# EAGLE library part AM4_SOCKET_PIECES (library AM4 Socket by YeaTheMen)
AM4 Socket Pins broken down into individual sections for convienience. Though it wasnt convientient for me as i spent hours making it >:I by yours truly, YeaTheMen
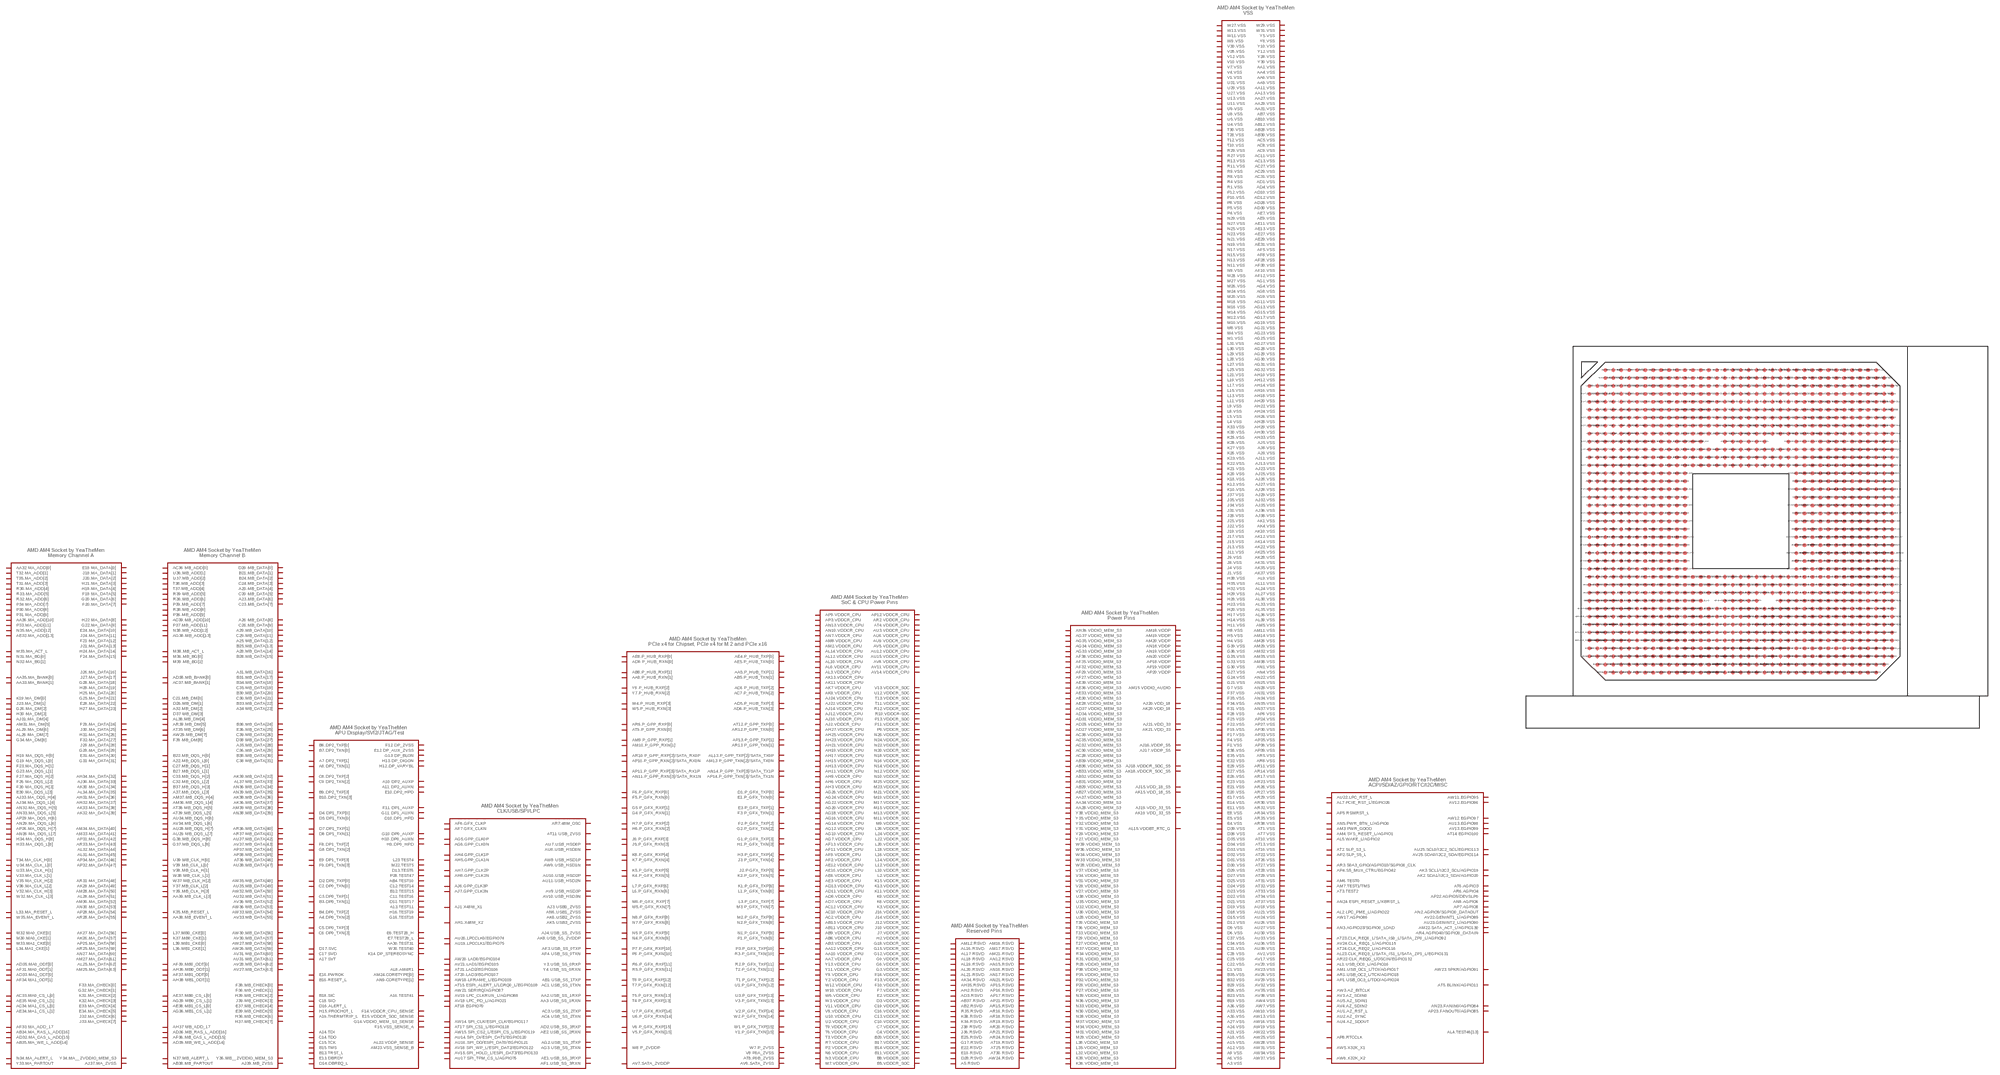
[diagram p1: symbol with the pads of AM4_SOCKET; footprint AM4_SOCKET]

Designator prefix -; gates G$1=AM4_SOCKET_MEM_A G$2=AM4_SOCKET_MEM_B G$3=AM4_SOCKET_CONTROL G$4=AM4_SOCKET_IO G$5=AM4_SOCKET_PCIE G$6=AM4_SOCKET_PWR G$7=AM4_SOCKET_RSVD G$8=AM4_SOCKET_VDD G$9=AM4_SOCKET_VSS G$10=AM4_SOCKET_MISC

## AM4_SOCKET_PIECES  [AM4_SOCKET]
A3.VSS  G$9:A3.VSS  out
A4.DP0_TXN[2]  G$3:A4.DP0_TXN[2]
A5.RSVD  G$7:A5.RSVD  nc
A6.VSS  G$9:A6.VSS  out
A7.DP2_TXP[1]  G$3:A7.DP2_TXP[1]
A8.DP2_TXN[1]  G$3:A8.DP2_TXN[1]
A9.VSS  G$9:A9.VSS  out
A10.DP2_AUXP  G$3:A10.DP2_AUXP
A11.DP2_AUXN  G$3:A11.DP2_AUXN
A12.VSS  G$9:A12.VSS  out
A13.TEST11  G$3:A13.TEST11
A14.TDI  G$3:A14.TDI
A15.VSS  G$9:A15.VSS  out
A16.TEST41  G$3:A16.TEST41
A17.SVT  G$3:A17.SVT
A18.VSS  G$9:A18.VSS  out
A19.THERMTRIP_L  G$3:A19.THERMTRIP_L
A20.MB_DATA[4]  G$2:A20.MB_DATA[4]
A21.VSS  G$9:A21.VSS  out
A22.MB_DQS_L[0]  G$2:A22.MB_DQS_L[0]
A23.MB_DATA[6]  G$2:A23.MB_DATA[6]
A24.VSS  G$9:A24.VSS  out
A25.MB_DATA[12]  G$2:A25.MB_DATA[12]
A26.MB_DATA[8]  G$2:A26.MB_DATA[8]
A27.VSS  G$9:A27.VSS  out
A28.MB_DATA[14]  G$2:A28.MB_DATA[14]
A29.MB_DATA[10]  G$2:A29.MB_DATA[10]
A30.VSS  G$9:A30.VSS  out
A31.MB_DATA[16]  G$2:A31.MB_DATA[16]
A32.MB_DM[2]  G$2:A32.MB_DM[2]
A33.VSS  G$9:A33.VSS  out
A34.MB_DATA[23]  G$2:A34.MB_DATA[23]
A35.MB_DATA[28]  G$2:A35.MB_DATA[28]
A36.VSS  G$9:A36.VSS  out
A37.MB_DQS_L[3]  G$2:A37.MB_DQS_L[3]
AA1.VSS  G$9:AA1.VSS  out
AA2.USB_SS_1RXP  G$4:AA2.USB_SS_1RXP
AA3.USB_SS_1RXN  G$4:AA3.USB_SS_1RXN
AA4.VSS  G$9:AA4.VSS  out
AA5.P_HUB_TXP[1]  G$5:AA5.P_HUB_TXP[1]
AA6.VSS  G$9:AA6.VSS  out
AA7.VDDCR_CPU  G$6:AA7.VDDCR_CPU  pwr
AA8.P_HUB_RXN[1]  G$5:AA8.P_HUB_RXN[1]
AA9.VSS  G$9:AA9.VSS  out
AA10.VDDCR_CPU  G$6:AA10.VDDCR_CPU  pwr
AA11.VSS  G$9:AA11.VSS  out
AA12.VDDCR_CPU  G$6:AA12.VDDCR_CPU  pwr
AA13.VSS  G$9:AA13.VSS  out
AA27.VSS  G$9:AA27.VSS  out
AA28.VDDIO_MEM_S3  G$8:AA28.VDDIO_MEM_S3  pwr
AA29.VSS  G$9:AA29.VSS  out
AA30.TEST31  G$3:AA30.TEST31
AA31.VSS  G$9:AA31.VSS  out
AA32.MA_ADD[0]  G$1:AA32.MA_ADD[0]
AA33.MA_BANK[1]  G$1:AA33.MA_BANK[1]
AA34.VDDIO_MEM_S3  G$8:AA34.VDDIO_MEM_S3  pwr
AA35.MA_BANK[0]  G$1:AA35.MA_BANK[0]
AA36.MA_ADD[10]  G$1:AA36.MA_ADD[10]
AA37.VDDIO_MEM_S3  G$8:AA37.VDDIO_MEM_S3  pwr
AA38.MB_EVENT_L  G$2:AA38.MB_EVENT_L
AA39.MB_CLK_L[3]  G$2:AA39.MB_CLK_L[3]
AB1.USB_SS_1TXP  G$4:AB1.USB_SS_1TXP
AB2.RSVD  G$7:AB2.RSVD  nc
AB3.VDDCR_CPU  G$6:AB3.VDDCR_CPU  pwr
AB4.TEST10  G$3:AB4.TEST10
AB5.P_HUB_TXN[1]  G$5:AB5.P_HUB_TXN[1]
AB6.VDDCR_CPU  G$6:AB6.VDDCR_CPU  pwr
AB7.VSS  G$9:AB7.VSS  out
AB8.P_HUB_RXP[1]  G$5:AB8.P_HUB_RXP[1]
AB9.VDDCR_CPU  G$6:AB9.VDDCR_CPU  pwr
AB10.VSS  G$9:AB10.VSS  out
AB11.VDDCR_CPU  G$6:AB11.VDDCR_CPU  pwr
AB12.VSS  G$9:AB12.VSS  out
AB13.VDDCR_CPU  G$6:AB13.VDDCR_CPU  pwr
AB27.VDDIO_MEM_S3  G$8:AB27.VDDIO_MEM_S3  pwr
AB28.VSS  G$9:AB28.VSS  out
AB29.VDDIO_MEM_S3  G$8:AB29.VDDIO_MEM_S3  pwr
AB30.VSS  G$9:AB30.VSS  out
AB31.VDDIO_MEM_S3  G$8:AB31.VDDIO_MEM_S3  pwr
AB32.VDDIO_MEM_S3  G$8:AB32.VDDIO_MEM_S3  pwr
AB33.VDDIO_MEM_S3  G$8:AB33.VDDIO_MEM_S3  pwr
AB34.MA_RAS_L_ADD[16]  G$1:AB34.MA_RAS_L_ADD[16]
AB35.MA_WE_L_ADD[14]  G$1:AB35.MA_WE_L_ADD[14]
AB36.VDDIO_MEM_S3  G$8:AB36.VDDIO_MEM_S3  pwr
AB37.RSVD  G$7:AB37.RSVD  nc
AB38.MB_PARTOUT  G$2:AB38.MB_PARTOUT  out
AB39.VDDIO_MEM_S3  G$8:AB39.VDDIO_MEM_S3  pwr
AC1.USB_SS_1TXN  G$4:AC1.USB_SS_1TXN
AC2.VDDCR_CPU  G$6:AC2.VDDCR_CPU  pwr
AC3.USB_SS_2TXP  G$4:AC3.USB_SS_2TXP
AC4.USB_SS_2TXN  G$4:AC4.USB_SS_2TXN
AC5.VSS  G$9:AC5.VSS  out
AC6.P_HUB_TXP[2]  G$5:AC6.P_HUB_TXP[2]
AC7.P_HUB_TXN[2]  G$5:AC7.P_HUB_TXN[2]
AC8.VSS  G$9:AC8.VSS  out
AC9.VSS  G$9:AC9.VSS  out
AC10.VDDCR_CPU  G$6:AC10.VDDCR_CPU  pwr
AC11.VSS  G$9:AC11.VSS  out
AC12.VDDCR_CPU  G$6:AC12.VDDCR_CPU  pwr
AC13.VSS  G$9:AC13.VSS  out
AC27.VSS  G$9:AC27.VSS  out
AC28.VDDIO_MEM_S3  G$8:AC28.VDDIO_MEM_S3  pwr
AC29.VSS  G$9:AC29.VSS  out
AC30.VDDIO_MEM_S3  G$8:AC30.VDDIO_MEM_S3  pwr
AC31.VSS  G$9:AC31.VSS  out
AC32.VDDIO_MEM_S3  G$8:AC32.VDDIO_MEM_S3  pwr
AC33.MA0_CS_L[0]  G$1:AC33.MA0_CS_L[0]
AC34.MA1_CS_L[0]  G$1:AC34.MA1_CS_L[0]
AC35.VDDIO_MEM_S3  G$8:AC35.VDDIO_MEM_S3  pwr
AC36.MB_ADD[0]  G$2:AC36.MB_ADD[0]
AC37.MB_BANK[1]  G$2:AC37.MB_BANK[1]
AC38.VDDIO_MEM_S3  G$8:AC38.VDDIO_MEM_S3  pwr
AC39.MB_ADD[10]  G$2:AC39.MB_ADD[10]
AD1.VSS  G$9:AD1.VSS  out
AD2.USB_SS_3RXP  G$4:AD2.USB_SS_3RXP
AD3.RSVD  G$7:AD3.RSVD  nc
AD4.VSS  G$9:AD4.VSS  out
AD5.P_HUB_TXP[3]  G$5:AD5.P_HUB_TXP[3]
AD6.P_HUB_TXN[3]  G$5:AD6.P_HUB_TXN[3]
AD7.VDDCR_CPU  G$6:AD7.VDDCR_CPU  pwr
AD8.P_HUB_RXN[0]  G$5:AD8.P_HUB_RXN[0]
AD9.VDDCR_CPU  G$6:AD9.VDDCR_CPU  pwr
AD10.VSS  G$9:AD10.VSS  out
AD11.VDDCR_CPU  G$6:AD11.VDDCR_CPU  pwr
AD12.VSS  G$9:AD12.VSS  out
AD13.VDDCR_CPU  G$6:AD13.VDDCR_CPU  pwr
AD27.VDDIO_MEM_S3  G$8:AD27.VDDIO_MEM_S3  pwr
AD28.VSS  G$9:AD28.VSS  out
AD29.VDDIO_MEM_S3  G$8:AD29.VDDIO_MEM_S3  pwr
AD30.VSS  G$9:AD30.VSS  out
AD31.VDDIO_MEM_S3  G$8:AD31.VDDIO_MEM_S3  pwr
AD32.MA_CAS_L_ADD[15]  G$1:AD32.MA_CAS_L_ADD[15]
AD33.MA1_ODT[0]  G$1:AD33.MA1_ODT[0]
AD34.VDDIO_MEM_S3  G$8:AD34.VDDIO_MEM_S3  pwr
AD35.MA0_ODT[0]  G$1:AD35.MA0_ODT[0]
AD36.MB_RAS_L_ADD[16]  G$2:AD36.MB_RAS_L_ADD[16]
AD37.VDDIO_MEM_S3  G$8:AD37.VDDIO_MEM_S3  pwr
AD38.MB_BANK[0]  G$2:AD38.MB_BANK[0]
AD39.MB_WE_L_ADD[14]  G$2:AD39.MB_WE_L_ADD[14]
AE1.USB_SS_3RXP  G$4:AE1.USB_SS_3RXP
AE2.USB_SS_2RXN  G$4:AE2.USB_SS_2RXN
AE3.VDDCR_CPU  G$6:AE3.VDDCR_CPU  pwr
AE4.P_HUB_TXP[0]  G$5:AE4.P_HUB_TXP[0]
AE5.P_HUB_TXN[0]  G$5:AE5.P_HUB_TXN[0]
AE6.VDDCR_CPU  G$6:AE6.VDDCR_CPU  pwr
AE7.VSS  G$9:AE7.VSS  out
AE8.P_HUB_RXP[0]  G$5:AE8.P_HUB_RXP[0]
AE9.VSS  G$9:AE9.VSS  out
AE10.VDDCR_CPU  G$6:AE10.VDDCR_CPU  pwr
AE11.VSS  G$9:AE11.VSS  out
AE12.VDDCR_CPU  G$6:AE12.VDDCR_CPU  pwr
AE13.VSS  G$9:AE13.VSS  out
AE27.VSS  G$9:AE27.VSS  out
AE28.VDDIO_MEM_S3  G$8:AE28.VDDIO_MEM_S3  pwr
AE29.VSS  G$9:AE29.VSS  out
AE30.VDDIO_MEM_S3  G$8:AE30.VDDIO_MEM_S3  pwr
AE31.VSS  G$9:AE31.VSS  out
AE32.MA_ADD[13]  G$1:AE32.MA_ADD[13]
AE33.VDDIO_MEM_S3  G$8:AE33.VDDIO_MEM_S3  pwr
AE34.MA1_CS_L[1]  G$1:AE34.MA1_CS_L[1]
AE35.MA0_CS_L[1]  G$1:AE35.MA0_CS_L[1]
AE36.VDDIO_MEM_S3  G$8:AE36.VDDIO_MEM_S3  pwr
AE37.MB0_CS_L[0]  G$2:AE37.MB0_CS_L[0]
AE38.MB1_CS_L[0]  G$2:AE38.MB1_CS_L[0]
AE39.VDDIO_MEM_S3  G$8:AE39.VDDIO_MEM_S3  pwr
AF1.USB_SS_3RXN  G$4:AF1.USB_SS_3RXN
AF2.VDDCR_CPU  G$6:AF2.VDDCR_CPU  pwr
AF3.USB_SS_0TXP  G$4:AF3.USB_SS_0TXP
AF4.USB_SS_0TXN  G$4:AF4.USB_SS_0TXN
AF5.VSS  G$9:AF5.VSS  out
AF6.GFX_CLKP  G$4:AF6.GFX_CLKP
AF7.GFX_CLKN  G$4:AF7.GFX_CLKN
AF8.VSS  G$9:AF8.VSS  out
AF9.VDDCR_CPU  G$6:AF9.VDDCR_CPU  pwr
AF10.VSS  G$9:AF10.VSS  out
AF11.VDDCR_CPU  G$6:AF11.VDDCR_CPU  pwr
AF12.VSS  G$9:AF12.VSS  out
AF13.VDDCR_CPU  G$6:AF13.VDDCR_CPU  pwr
AF27.VDDIO_MEM_S3  G$8:AF27.VDDIO_MEM_S3  pwr
AF28.VSS  G$9:AF28.VSS  out
AF29.VDDIO_MEM_S3  G$8:AF29.VDDIO_MEM_S3  pwr
AF30.VSS  G$9:AF30.VSS  out
AF31.MA0_ODT[1]  G$1:AF31.MA0_ODT[1]
AF32.VDDIO_MEM_S3  G$8:AF32.VDDIO_MEM_S3  pwr
AF33.MA_ADD_17  G$1:AF33.MA_ADD_17
AF34.MA1_ODT[1]  G$1:AF34.MA1_ODT[1]
AF35.VDDIO_MEM_S3  G$8:AF35.VDDIO_MEM_S3  pwr
AF36.MB_CAS_L_ADD[15]  G$2:AF36.MB_CAS_L_ADD[15]
AF37.MB1_ODT[0]  G$2:AF37.MB1_ODT[0]
AF38.VDDIO_MEM_S3  G$8:AF38.VDDIO_MEM_S3  pwr
AF39.MB0_ODT[0]  G$2:AF39.MB0_ODT[0]
AG1.VSS  G$9:AG1.VSS  out
AG2.USB_SS_3TXP  G$4:AG2.USB_SS_3TXP
AG3.USB_SS_3TXN  G$4:AG3.USB_SS_3TXN
AG4.VSS  G$9:AG4.VSS  out
AG5.GPP_CLK0P  G$4:AG5.GPP_CLK0P
AG6.GPP_CLK0N  G$4:AG6.GPP_CLK0N
AG7.VDDCR_CPU  G$6:AG7.VDDCR_CPU  pwr
AG8.VSS  G$9:AG8.VSS  out
AG9.VSS  G$9:AG9.VSS  out
AG10.VDDCR_CPU  G$6:AG10.VDDCR_CPU  pwr
AG11.VSS  G$9:AG11.VSS  out
AG12.VDDCR_CPU  G$6:AG12.VDDCR_CPU  pwr
AG13.VSS  G$9:AG13.VSS  out
AG14.VDDCR_CPU  G$6:AG14.VDDCR_CPU  pwr
AG15.VSS  G$9:AG15.VSS  out
AG16.VDDCR_CPU  G$6:AG16.VDDCR_CPU  pwr
AG17.VSS  G$9:AG17.VSS  out
AG18.VDDCR_CPU  G$6:AG18.VDDCR_CPU  pwr
AG19.VSS  G$9:AG19.VSS  out
AG20.VDDCR_CPU  G$6:AG20.VDDCR_CPU  pwr
AG21.VSS  G$9:AG21.VSS  out
AG22.VDDCR_CPU  G$6:AG22.VDDCR_CPU  pwr
AG23.VSS  G$9:AG23.VSS  out
AG24.VDDCR_CPU  G$6:AG24.VDDCR_CPU  pwr
AG25.VSS  G$9:AG25.VSS  out
AG26.VDDCR_CPU  G$6:AG26.VDDCR_CPU  pwr
AG27.VSS  G$9:AG27.VSS  out
AG28.VSS  G$9:AG28.VSS  out
AG29.VSS  G$9:AG29.VSS  out
AG30.VSS  G$9:AG30.VSS  out
AG31.VSS  G$9:AG31.VSS  out
AG32.VSS  G$9:AG32.VSS  out
AG33.VDDIO_MEM_S3  G$8:AG33.VDDIO_MEM_S3  pwr
AG34.VDDIO_MEM_S3  G$8:AG34.VDDIO_MEM_S3  pwr
AG35.VDDIO_MEM_S3  G$8:AG35.VDDIO_MEM_S3  pwr
AG36.MB1_CS_L[1]  G$2:AG36.MB1_CS_L[1]
AG37.VDDIO_MEM_S3  G$8:AG37.VDDIO_MEM_S3  pwr
AG38.MB_ADD[13]  G$2:AG38.MB_ADD[13]
AG39.MB0_CS_L[1]  G$2:AG39.MB0_CS_L[1]
AH1.X48M_X2  G$4:AH1.X48M_X2
AH2.RSVD  G$7:AH2.RSVD  nc
AH3.VDDCR_CPU  G$6:AH3.VDDCR_CPU  pwr
AH4.GPP_CLK1P  G$4:AH4.GPP_CLK1P
AH5.GPP_CLK1N  G$4:AH5.GPP_CLK1N
AH6.VDDCR_CPU  G$6:AH6.VDDCR_CPU  pwr
AH7.GPP_CLK2P  G$4:AH7.GPP_CLK2P
AH8.GPP_CLK2N  G$4:AH8.GPP_CLK2N
AH9.VDDCR_CPU  G$6:AH9.VDDCR_CPU  pwr
AH10.VSS  G$9:AH10.VSS  out
AH11.VDDCR_CPU  G$6:AH11.VDDCR_CPU  pwr
AH12.VSS  G$9:AH12.VSS  out
AH13.VDDCR_CPU  G$6:AH13.VDDCR_CPU  pwr
AH14.VSS  G$9:AH14.VSS  out
AH15.VDDCR_CPU  G$6:AH15.VDDCR_CPU  pwr
AH16.VSS  G$9:AH16.VSS  out
AH17.VDDCR_CPU  G$6:AH17.VDDCR_CPU  pwr
AH18.VSS  G$9:AH18.VSS  out
AH19.VDDCR_CPU  G$6:AH19.VDDCR_CPU  pwr
AH20.VSS  G$9:AH20.VSS  out
AH21.VDDCR_CPU  G$6:AH21.VDDCR_CPU  pwr
AH22.VSS  G$9:AH22.VSS  out
AH23.VDDCR_CPU  G$6:AH23.VDDCR_CPU  pwr
AH24.VSS  G$9:AH24.VSS  out
AH25.VDDCR_CPU  G$6:AH25.VDDCR_CPU  pwr
AH26.VSS  G$9:AH26.VSS  out
AH27.VDDCR_CPU  G$6:AH27.VDDCR_CPU  pwr
AH28.VSS  G$9:AH28.VSS  out
AH29.VSS  G$9:AH29.VSS  out
AH30.VSS  G$9:AH30.VSS  out
AH31.MA_DATA[36]  G$1:AH31.MA_DATA[36]
AH32.MA_DATA[37]  G$1:AH32.MA_DATA[37]
AH33.VSS  G$9:AH33.VSS  out
AH34.MA_DATA[32]  G$1:AH34.MA_DATA[32]
AH35.RSVD  G$7:AH35.RSVD  nc
AH36.MB0_ODT[1]  G$2:AH36.MB0_ODT[1]
AH37.MB_ADD_17  G$2:AH37.MB_ADD_17
AH38.MB1_ODT[1]  G$2:AH38.MB1_ODT[1]
AH39.VDDIO_MEM_S3  G$8:AH39.VDDIO_MEM_S3  pwr
AJ1.X48M_X1  G$4:AJ1.X48M_X1
AJ2.VDDCR_CPU  G$6:AJ2.VDDCR_CPU  pwr
AJ3.USB0_ZVSS  G$4:AJ3.USB0_ZVSS  out
AJ4.USB_SS_ZVSS  G$4:AJ4.USB_SS_ZVSS  out
AJ5.VSS  G$9:AJ5.VSS  out
AJ6.GPP_CLK3P  G$4:AJ6.GPP_CLK3P
AJ7.GPP_CLK3N  G$4:AJ7.GPP_CLK3N
AJ8.VSS  G$9:AJ8.VSS  out
AJ9.VSS  G$9:AJ9.VSS  out
AJ10.VDDCR_CPU  G$6:AJ10.VDDCR_CPU  pwr
AJ11.VSS  G$9:AJ11.VSS  out
AJ12.VDDCR_CPU  G$6:AJ12.VDDCR_CPU  pwr
AJ13.VSS  G$9:AJ13.VSS  out
AJ14.VDDCR_CPU  G$6:AJ14.VDDCR_CPU  pwr
AJ15.VDD_18_S5  G$8:AJ15.VDD_18_S5  pwr
AJ16.VDDP_S5  G$8:AJ16.VDDP_S5  pwr
AJ17.VDDP_S5  G$8:AJ17.VDDP_S5  pwr
AJ18.VDDCR_SOC_S5  G$8:AJ18.VDDCR_SOC_S5  pwr
AJ19.VDD_33_S5  G$8:AJ19.VDD_33_S5  pwr
AJ20.VDD_18  G$8:AJ20.VDD_18  pwr
AJ21.VDD_33  G$8:AJ21.VDD_33  pwr
AJ22.VDDCR_CPU  G$6:AJ22.VDDCR_CPU  pwr
AJ23.VSS  G$9:AJ23.VSS  out
AJ24.VDDCR_CPU  G$6:AJ24.VDDCR_CPU  pwr
AJ25.VSS  G$9:AJ25.VSS  out
AJ26.VSS  G$9:AJ26.VSS  out
AJ27.VSS  G$9:AJ27.VSS  out
AJ28.VSS  G$9:AJ28.VSS  out
AJ29.VSS  G$9:AJ29.VSS  out
AJ30.MA_DATA[33]  G$1:AJ30.MA_DATA[33]
AJ31.MA_DM[4]  G$1:AJ31.MA_DM[4]
AJ32.VSS  G$9:AJ32.VSS  out
AJ33.MA_DQS_H[4]  G$1:AJ33.MA_DQS_H[4]
AJ34.MA_DQS_L[4]  G$1:AJ34.MA_DQS_L[4]
AJ35.VSS  G$9:AJ35.VSS  out
AJ36.VSS  G$9:AJ36.VSS  out
AJ37.MA_ZVSS  G$1:AJ37.MA_ZVSS  out
AJ38.VSS  G$9:AJ38.VSS  out
AJ39.MB_ZVSS  G$2:AJ39.MB_ZVSS  out
AK1.VSS  G$9:AK1.VSS  out
AK2.SDA1/I2C3_SDA/AGPIO20  G$10:AK2.SDA1/I2C3_SDA/AGPIO20
AK3.SCL1/I2C3_SCL/AGPIO19  G$10:AK3.SCL1/I2C3_SCL/AGPIO19
AK4.VSS  G$9:AK4.VSS  out
AK5.USB3_ZVSS  G$4:AK5.USB3_ZVSS  out
AK6.USB2_ZVSS  G$4:AK6.USB2_ZVSS  out
AK7.VDDCR_CPU  G$6:AK7.VDDCR_CPU  pwr
AK8.USB_SS_ZVDDP  G$4:AK8.USB_SS_ZVDDP  pwr
AK9.VDDCR_CPU  G$6:AK9.VDDCR_CPU  pwr
AK10.VSS  G$9:AK10.VSS  out
AK11.VDDCR_CPU  G$6:AK11.VDDCR_CPU  pwr
AK12.VSS  G$9:AK12.VSS  out
AK13.VDDCR_CPU  G$6:AK13.VDDCR_CPU  pwr
AK14.VSS  G$9:AK14.VSS  out
AK15.VDD_18_S5  G$8:AK15.VDD_18_S5  pwr
AK18.VDDCR_SOC_S5  G$8:AK18.VDDCR_SOC_S5  pwr
AK19.VDD_33_S5  G$8:AK19.VDD_33_S5  pwr
AK20.VDD_18  G$8:AK20.VDD_18  pwr
AK21.VDD_33  G$8:AK21.VDD_33  pwr
AK22.VSS  G$9:AK22.VSS  out
AK25.VSS  G$9:AK25.VSS  out
AK26.MA_DATA[57]  G$1:AK26.MA_DATA[57]
AK27.MA_DATA[56]  G$1:AK27.MA_DATA[56]
AK28.VSS  G$9:AK28.VSS  out
AK29.MA_DATA[49]  G$1:AK29.MA_DATA[49]
AK30.MA_DATA[34]  G$1:AK30.MA_DATA[34]
AK31.VSS  G$9:AK31.VSS  out
AK32.MA_DATA[39]  G$1:AK32.MA_DATA[39]
AK33.MA_DATA[38]  G$1:AK33.MA_DATA[38]
AK34.RSVD  G$7:AK34.RSVD  nc
AK35.VSS  G$9:AK35.VSS  out
AK36.MB_DATA[37]  G$2:AK36.MB_DATA[37]
AK37.VSS  G$9:AK37.VSS  out
AK38.MB_DATA[36]  G$2:AK38.MB_DATA[36]
AK39.MB_DATA[32]  G$2:AK39.MB_DATA[32]
AL1.USB_OC0_L/AGPIO16  G$10:AL1.USB_OC0_L/AGPIO16
AL2.LPC_PME_L/AGPIO22  G$10:AL2.LPC_PME_L/AGPIO22
AL3.VDDCR_CPU  G$6:AL3.VDDCR_CPU  pwr
AL4.TEST46[13]  G$10:AL4.TEST46[13]
AL5.WAKE_L/AGPIO2  G$10:AL5.WAKE_L/AGPIO2
AL6.VDDCR_CPU  G$6:AL6.VDDCR_CPU  pwr
AL7.PCIE_RST_L/EGPIO26  G$10:AL7.PCIE_RST_L/EGPIO26
AL8.AM4R1  G$3:AL8.AM4R1
AL9.VSS  G$9:AL9.VSS  out
AL10.VDDCR_CPU  G$6:AL10.VDDCR_CPU  pwr
AL11.VSS  G$9:AL11.VSS  out
AL12.VDDCR_CPU  G$6:AL12.VDDCR_CPU  pwr
AL13.P_GPP_TXP[2]/SATA_TX0P  G$5:AL13.P_GPP_TXP[2]/SATA_TX0P
AL14.VDDCR_CPU  G$6:AL14.VDDCR_CPU  pwr
AL15.VDDBT_RTC_G  G$8:AL15.VDDBT_RTC_G  pwr
AL16.RSVD  G$7:AL16.RSVD  nc
AL17.RSVD  G$7:AL17.RSVD  nc
AL18.RSVD  G$7:AL18.RSVD  nc
AL19.RSVD  G$7:AL19.RSVD  nc
AL20.RSVD  G$7:AL20.RSVD  nc
AL21.RSVD  G$7:AL21.RSVD  nc
AL22.VDDP_SENSE  G$3:AL22.VDDP_SENSE  pwr
AL23.CLK_REQ3_L/SATA_IS1_L/SATA_ZP1_L/EGPIO131  G$10:AL23.CLK_REQ3_L/SATA_IS1_L/SATA_ZP1_L/EGPIO131
AL24.VSS  G$9:AL24.VSS  out
AL25.MA_DATA[62]  G$1:AL25.MA_DATA[62]
AL26.MA_DM[7]  G$1:AL26.MA_DM[7]
AL27.VSS  G$9:AL27.VSS  out
AL28.MA_DATA[51]  G$1:AL28.MA_DATA[51]
AL29.MA_DM[6]  G$1:AL29.MA_DM[6]
AL30.VSS  G$9:AL30.VSS  out
AL31.MA_DATA[45]  G$1:AL31.MA_DATA[45]
AL32.MA_DATA[44]  G$1:AL32.MA_DATA[44]
AL33.VSS  G$9:AL33.VSS  out
AL34.MA_DATA[35]  G$1:AL34.MA_DATA[35]
AL35.VSS  G$9:AL35.VSS  out
AL36.VSS  G$9:AL36.VSS  out
AL37.MB_DATA[33]  G$2:AL37.MB_DATA[33]
AL38.MB_DM[4]  G$2:AL38.MB_DM[4]
AL39.VSS  G$9:AL39.VSS  out
AM1.USB_OC1_L/TDI/AGPIO17  G$10:AM1.USB_OC1_L/TDI/AGPIO17
AM2.VDDCR_CPU  G$6:AM2.VDDCR_CPU  pwr
AM3.PWR_GOOD  G$10:AM3.PWR_GOOD
AM4.SYS_RESET_L/AGPIO1  G$10:AM4.SYS_RESET_L/AGPIO1
AM5.VSS  G$9:AM5.VSS  out
AM6.TEST0  G$10:AM6.TEST0
AM7.TEST1/TMS  G$10:AM7.TEST1/TMS
AM8.VDDCR_CPU  G$6:AM8.VDDCR_CPU  pwr
AM9.P_GPP_RXP[1]  G$5:AM9.P_GPP_RXP[1]
AM10.P_GPP_RXN[1]  G$5:AM10.P_GPP_RXN[1]
AM11.VSS  G$9:AM11.VSS  out
AM12.RSVD  G$7:AM12.RSVD  nc
AM13.P_GPP_TXN[2]/SATA_TX0N  G$5:AM13.P_GPP_TXN[2]/SATA_TX0N
AM14.VSS  G$9:AM14.VSS  out
AM15.VDDIO_AUDIO  G$8:AM15.VDDIO_AUDIO  pwr
AM16.RSVD  G$7:AM16.RSVD  nc
AM17.RSVD  G$7:AM17.RSVD  nc
AM18.VDDP  G$8:AM18.VDDP  pwr
AM19.VDDP  G$8:AM19.VDDP  pwr
AM20.VDDP  G$8:AM20.VDDP  pwr
AM21.RSVD  G$7:AM21.RSVD  nc
AM22.SATA_ACT_L/AGPIO130  G$10:AM22.SATA_ACT_L/AGPIO130
AM23.VSS_SENSE_B  G$3:AM23.VSS_SENSE_B
AM24.CORETYPE[0]  G$3:AM24.CORETYPE[0]
AM25.MA_DATA[63]  G$1:AM25.MA_DATA[63]
AM26.VSS  G$9:AM26.VSS  out
AM27.MA_DATA[61]  G$1:AM27.MA_DATA[61]
AM28.MA_DATA[50]  G$1:AM28.MA_DATA[50]
AM29.VSS  G$9:AM29.VSS  out
AM30.MA_DATA[52]  G$1:AM30.MA_DATA[52]
AM31.MA_DM[5]  G$1:AM31.MA_DM[5]
AM32.VSS  G$9:AM32.VSS  out
AM33.MA_DATA[41]  G$1:AM33.MA_DATA[41]
AM34.MA_DATA[40]  G$1:AM34.MA_DATA[40]
AM35.VSS  G$9:AM35.VSS  out
AM36.MB_DQS_L[4]  G$2:AM36.MB_DQS_L[4]
AM37.MB_DQS_H[4]  G$2:AM37.MB_DQS_H[4]
AM38.VSS  G$9:AM38.VSS  out
AM39.MB_DATA[38]  G$2:AM39.MB_DATA[38]
AN1.VSS  G$9:AN1.VSS  out
AN2.AGPIO9/SGPIO0_DATAOUT  G$10:AN2.AGPIO9/SGPIO0_DATAOUT  out
AN3.AGPIO23/SGPIO0_LOAD  G$10:AN3.AGPIO23/SGPIO0_LOAD
AN4.VSS  G$9:AN4.VSS  out
AN5.PWR_BTN_L/AGPIO0  G$10:AN5.PWR_BTN_L/AGPIO0
AN6.USB1_ZVSS  G$4:AN6.USB1_ZVSS  out
AN7.VDDCR_CPU  G$6:AN7.VDDCR_CPU  pwr
AN8.AGPIO6  G$10:AN8.AGPIO6
AN9.CORETYPE[1]  G$3:AN9.CORETYPE[1]
AN10.VDDCR_CPU  G$6:AN10.VDDCR_CPU  pwr
AN11.P_GPP_RXN[3]/SATA_RX1N  G$5:AN11.P_GPP_RXN[3]/SATA_RX1N
AN12.RSVD  G$7:AN12.RSVD  nc
AN13.VDDCR_CPU  G$6:AN13.VDDCR_CPU  pwr
AN14.P_GPP_TXP[3]/SATA_TX1P  G$5:AN14.P_GPP_TXP[3]/SATA_TX1P
AN15.RSVD  G$7:AN15.RSVD  nc
AN16.RSVD  G$7:AN16.RSVD  nc
AN17.RSVD  G$7:AN17.RSVD  nc
AN18.VDDP  G$8:AN18.VDDP  pwr
AN19.VDDP  G$8:AN19.VDDP  pwr
AN20.VDDP  G$8:AN20.VDDP  pwr
AN21.RSVD  G$7:AN21.RSVD  nc
AN22.VSS  G$9:AN22.VSS  out
AN23.FANIN0/AGPIO84  G$10:AN23.FANIN0/AGPIO84  in
AN24.ESPI_RESET_L/KBRST_L  G$10:AN24.ESPI_RESET_L/KBRST_L
AN25.VSS  G$9:AN25.VSS  out
AN26.MA_DQS_L[7]  G$1:AN26.MA_DQS_L[7]
AN27.MA_DATA[60]  G$1:AN27.MA_DATA[60]
AN28.VSS  G$9:AN28.VSS  out
AN29.MA_DQS_L[6]  G$1:AN29.MA_DQS_L[6]
AN30.MA_DATA[53]  G$1:AN30.MA_DATA[53]
AN31.VSS  G$9:AN31.VSS  out
AN32.MA_DQS_H[5]  G$1:AN32.MA_DQS_H[5]
AN33.MA_DQS_L[5]  G$1:AN33.MA_DQS_L[5]
AN34.VSS  G$9:AN34.VSS  out
AN35.VSS  G$9:AN35.VSS  out
AN36.MB_DATA[34]  G$2:AN36.MB_DATA[34]
AN37.VSS  G$9:AN37.VSS  out
AN38.MB_DATA[39]  G$2:AN38.MB_DATA[39]
AN39.MB_DATA[35]  G$2:AN39.MB_DATA[35]
AP1.USB_OC3_L/TDO/AGPIO24  G$10:AP1.USB_OC3_L/TDO/AGPIO24
AP2.SLP_S5_L  G$10:AP2.SLP_S5_L
AP3.VDDCR_CPU  G$6:AP3.VDDCR_CPU  pwr
AP4.S5_MUX_CTRL/EGPIO42  G$10:AP4.S5_MUX_CTRL/EGPIO42
AP5.RSMRST_L  G$10:AP5.RSMRST_L
AP6.VSS  G$9:AP6.VSS  out
AP7.AGPIO8  G$10:AP7.AGPIO8
AP8.RTCCLK  G$10:AP8.RTCCLK
AP9.VDDCR_CPU  G$6:AP9.VDDCR_CPU  pwr
AP10.P_GPP_RXN[2]/SATA_RX0N  G$5:AP10.P_GPP_RXN[2]/SATA_RX0N
AP11.P_GPP_RXP[3]/SATA_RX1P  G$5:AP11.P_GPP_RXP[3]/SATA_RX1P
AP12.VDDCR_CPU  G$6:AP12.VDDCR_CPU  pwr
AP13.P_GPP_TXP[1]  G$5:AP13.P_GPP_TXP[1]
AP14.P_GPP_TXN[3]/SATA_TX1N  G$5:AP14.P_GPP_TXN[3]/SATA_TX1N
AP15.RSVD  G$7:AP15.RSVD  nc
AP16.RSVD  G$7:AP16.RSVD  nc
AP17.RSVD  G$7:AP17.RSVD  nc
AP18.VDDP  G$8:AP18.VDDP  pwr
AP19.VDDP  G$8:AP19.VDDP  pwr
AP20.VDDP  G$8:AP20.VDDP  pwr
AP21.RSVD  G$7:AP21.RSVD  nc
AP22.AGPIO5/DEVSLP0  G$10:AP22.AGPIO5/DEVSLP0
AP23.FANOUT0/AGPIO85  G$10:AP23.FANOUT0/AGPIO85  out
AP24.VSS  G$9:AP24.VSS  out
AP25.MA_DATA[58]  G$1:AP25.MA_DATA[58]
AP26.MA_DQS_H[7]  G$1:AP26.MA_DQS_H[7]
AP27.VSS  G$9:AP27.VSS  out
AP28.MA_DATA[54]  G$1:AP28.MA_DATA[54]
AP29.MA_DQS_H[6]  G$1:AP29.MA_DQS_H[6]
AP30.VSS  G$9:AP30.VSS  out
AP31.MA_DATA[42]  G$1:AP31.MA_DATA[42]
AP32.MA_DATA[47]  G$1:AP32.MA_DATA[47]
AP33.VSS  G$9:AP33.VSS  out
AP34.MA_DATA[46]  G$1:AP34.MA_DATA[46]
AP35.VSS  G$9:AP35.VSS  out
AP36.VSS  G$9:AP36.VSS  out
AP37.MB_DATA[44]  G$2:AP37.MB_DATA[44]
AP38.MB_DATA[45]  G$2:AP38.MB_DATA[45]
AP39.VSS  G$9:AP39.VSS  out
AR1.USB_OC2_L/TCK/AGPIO18  G$10:AR1.USB_OC2_L/TCK/AGPIO18
AR2.VDDCR_CPU  G$6:AR2.VDDCR_CPU  pwr
AR3.S0A3_GPIO/AGPIO10/SGPIO0_CLK  G$10:AR3.S0A3_GPIO/AGPIO10/SGPIO0_CLK
AR4.AGPIO40/SGPIO0_DATAIN  G$10:AR4.AGPIO40/SGPIO0_DATAIN  in
AR5.VSS  G$9:AR5.VSS  out
AR6.AGPIO4  G$10:AR6.AGPIO4
AR7.48M_OSC  G$4:AR7.48M_OSC
AR8.VSS  G$9:AR8.VSS  out
AR9.P_GPP_RXP[0]  G$5:AR9.P_GPP_RXP[0]
AR10.P_GPP_RXP[2]/SATA_RX0P  G$5:AR10.P_GPP_RXP[2]/SATA_RX0P
AR11.VSS  G$9:AR11.VSS  out
AR12.P_GPP_TXN[0]  G$5:AR12.P_GPP_TXN[0]
AR13.P_GPP_TXN[1]  G$5:AR13.P_GPP_TXN[1]
AR14.VSS  G$9:AR14.VSS  out
AR15.RSVD  G$7:AR15.RSVD  nc
AR16.RSVD  G$7:AR16.RSVD  nc
AR17.VSS  G$9:AR17.VSS  out
AR18.RSVD  G$7:AR18.RSVD  nc
AR19.RSVD  G$7:AR19.RSVD  nc
AR20.RSVD  G$7:AR20.RSVD  nc
AR21.RSVD  G$7:AR21.RSVD  nc
AR22.CLK_REQG_L/OSCIN/EGPIO132  G$10:AR22.CLK_REQG_L/OSCIN/EGPIO132  in
AR23.VSS  G$9:AR23.VSS  out
AR24.RSVD  G$7:AR24.RSVD  nc
AR25.MA_DATA[59]  G$1:AR25.MA_DATA[59]
AR26.VSS  G$9:AR26.VSS  out
AR27.VSS  G$9:AR27.VSS  out
AR28.MA_DATA[55]  G$1:AR28.MA_DATA[55]
AR29.VSS  G$9:AR29.VSS  out
AR30.VSS  G$9:AR30.VSS  out
AR31.MA_DATA[48]  G$1:AR31.MA_DATA[48]
AR32.VSS  G$9:AR32.VSS  out
AR33.MA_DATA[43]  G$1:AR33.MA_DATA[43]
AR34.VSS  G$9:AR34.VSS  out
AR35.VSS  G$9:AR35.VSS  out
AR36.MB_DATA[40]  G$2:AR36.MB_DATA[40]
AR37.MB_DATA[41]  G$2:AR37.MB_DATA[41]
AR38.VSS  G$9:AR38.VSS  out
AR39.MB_DM[5]  G$2:AR39.MB_DM[5]
AT1.VSS  G$9:AT1.VSS  out
AT2.SLP_S3_L  G$10:AT2.SLP_S3_L
AT3.TEST2  G$10:AT3.TEST2
AT4.VDDCR_CPU  G$6:AT4.VDDCR_CPU  pwr
AT5.BLINK/AGPIO11  G$10:AT5.BLINK/AGPIO11  in
AT6.AGPIO3  G$10:AT6.AGPIO3
AT7.VSS  G$9:AT7.VSS  out
AT8.P0B_ZVSS  G$5:AT8.P0B_ZVSS  out
AT9.P_GPP_RXN[0]  G$5:AT9.P_GPP_RXN[0]
AT10.VSS  G$9:AT10.VSS  out
AT11.USB_ZVSS  G$4:AT11.USB_ZVSS  out
AT12.P_GPP_TXP[0]  G$5:AT12.P_GPP_TXP[0]
AT13.VSS  G$9:AT13.VSS  out
AT14.EGPIO100  G$10:AT14.EGPIO100
AT15.ESPI_ALERT_L/LDRQ0_L/EGPIO108  G$4:AT15.ESPI_ALERT_L/LDRQ0_L/EGPIO108
AT16.VSS  G$9:AT16.VSS  out
AT17.SPI_CS1_L/EGPIO118  G$4:AT17.SPI_CS1_L/EGPIO118
AT18.EGPIO70  G$4:AT18.EGPIO70
AT19.RSVD  G$7:AT19.RSVD  nc
AT20.LAD3/EGPIO107  G$4:AT20.LAD3/EGPIO107
AT21.LAD2/EGPIO106  G$4:AT21.LAD2/EGPIO106
AT22.VSS  G$9:AT22.VSS  out
AT23.CLK_REQ0_L/SATA_IS0_L/SATA_ZP0_L/AGPIO92  G$10:AT23.CLK_REQ0_L/SATA_IS0_L/SATA_ZP0_L/AGPIO92
AT24.CLK_REQ2_L/AGPIO116  G$10:AT24.CLK_REQ2_L/AGPIO116
AT25.RSVD  G$7:AT25.RSVD  nc
AT26.VSS  G$9:AT26.VSS  out
AT27.VSS  G$9:AT27.VSS  out
AT28.VSS  G$9:AT28.VSS  out
AT29.VSS  G$9:AT29.VSS  out
AT30.RSVD  G$7:AT30.RSVD  nc
AT31.VSS  G$9:AT31.VSS  out
AT32.VSS  G$9:AT32.VSS  out
AT33.VSS  G$9:AT33.VSS  out
AT34.VSS  G$9:AT34.VSS  out
AT35.MB_DM[6]  G$2:AT35.MB_DM[6]
AT36.MB_DATA[46]  G$2:AT36.MB_DATA[46]
AT37.VSS  G$9:AT37.VSS  out
AT38.MB_DQS_H[5]  G$2:AT38.MB_DQS_H[5]
AT39.MB_DQS_L[5]  G$2:AT39.MB_DQS_L[5]
AU1.AZ_RST_L  G$10:AU1.AZ_RST_L
AU2.AZ_SYNC  G$10:AU2.AZ_SYNC
AU3.VDDCR_CPU  G$6:AU3.VDDCR_CPU  pwr
AU4.AZ_SDOUT  G$10:AU4.AZ_SDOUT  out
AU5.AZ_SDIN1  G$10:AU5.AZ_SDIN1  in
AU6.VDDCR_CPU  G$6:AU6.VDDCR_CPU  pwr
AU7.USB_HSD0P  G$4:AU7.USB_HSD0P
AU8.USB_HSD0N  G$4:AU8.USB_HSD0N
AU9.VDDCR_CPU  G$6:AU9.VDDCR_CPU  pwr
AU10.USB_HSD2P  G$4:AU10.USB_HSD2P
AU11.USB_HSD2N  G$4:AU11.USB_HSD2N
AU12.VDDCR_CPU  G$6:AU12.VDDCR_CPU  pwr
AU13.EGPIO98  G$10:AU13.EGPIO98
AU14.SPI_DI/ESPI_DAT1/EGPIO120  G$4:AU14.SPI_DI/ESPI_DAT1/EGPIO120
AU15.VDDCR_CPU  G$6:AU15.VDDCR_CPU  pwr
AU16.SPI_DO/ESPI_DAT0/EGPIO121  G$4:AU16.SPI_DO/ESPI_DAT0/EGPIO121
AU17.SPI_TPM_CS_L/AGPIO76  G$4:AU17.SPI_TPM_CS_L/AGPIO76
AU18.VSS  G$9:AU18.VSS  out
AU19.LPCCLK1/EGPIO75  G$4:AU19.LPCCLK1/EGPIO75
AU20.LPCCLK0/EGPIO74  G$4:AU20.LPCCLK0/EGPIO74
AU21.VSS  G$9:AU21.VSS  out
AU22.LPC_RST_L  G$10:AU22.LPC_RST_L
AU23.GENINT2_L/AGPIO90  G$10:AU23.GENINT2_L/AGPIO90  in
AU24.VSS  G$9:AU24.VSS  out
AU25.SCL0/I2C2_SCL/EGPIO113  G$10:AU25.SCL0/I2C2_SCL/EGPIO113
AU26.VSS  G$9:AU26.VSS  out
AU27.VSS  G$9:AU27.VSS  out
AU28.MB_DQS_H[7]  G$2:AU28.MB_DQS_H[7]
AU29.MB_DQS_L[7]  G$2:AU29.MB_DQS_L[7]
AU30.VSS  G$9:AU30.VSS  out
AU31.MB_DATA[61]  G$2:AU31.MB_DATA[61]
AU32.MB_DATA[51]  G$2:AU32.MB_DATA[51]
AU33.VSS  G$9:AU33.VSS  out
AU34.MB_DQS_H[6]  G$2:AU34.MB_DQS_H[6]
AU35.MB_DATA[49]  G$2:AU35.MB_DATA[49]
AU36.VSS  G$9:AU36.VSS  out
AU37.MB_DATA[42]  G$2:AU37.MB_DATA[42]
AU38.MB_DATA[47]  G$2:AU38.MB_DATA[47]
AU39.VSS  G$9:AU39.VSS  out
AV2.VSS  G$9:AV2.VSS  out
AV3.AZ_SDIN0  G$10:AV3.AZ_SDIN0  in
AV4.AZ_SDIN2  G$10:AV4.AZ_SDIN2  in
AV5.VDDCR_CPU  G$6:AV5.VDDCR_CPU  pwr
AV6.SATA_ZVSS  G$5:AV6.SATA_ZVSS  out
AV7.SATA_ZVDDP  G$5:AV7.SATA_ZVDDP  pwr
AV8.VDDCR_CPU  G$6:AV8.VDDCR_CPU  pwr
AV9.USB_HSD3P  G$4:AV9.USB_HSD3P
AV10.USB_HSD3N  G$4:AV10.USB_HSD3N
AV11.VDDCR_CPU  G$6:AV11.VDDCR_CPU  pwr
AV12.EGPIO96  G$10:AV12.EGPIO96
AV13.EGPIO99  G$10:AV13.EGPIO99
AV14.VDDCR_CPU  G$6:AV14.VDDCR_CPU  pwr
AV15.SPI_HOLD_L/ESPI_DAT3/EGPIO133  G$4:AV15.SPI_HOLD_L/ESPI_DAT3/EGPIO133
AV16.SPI_WP_L/ESPI_DAT2/EGPIO122  G$4:AV16.SPI_WP_L/ESPI_DAT2/EGPIO122
AV17.VSS  G$9:AV17.VSS  out
AV18.LPC_PD_L/AGPIO21  G$4:AV18.LPC_PD_L/AGPIO21
AV19.LPC_CLKRUN_L/AGPIO88  G$4:AV19.LPC_CLKRUN_L/AGPIO88
AV20.VSS  G$9:AV20.VSS  out
AV21.LAD1/EGPIO105  G$4:AV21.LAD1/EGPIO105
AV22.GENINT1_L/AGPIO89  G$10:AV22.GENINT1_L/AGPIO89  in
AV23.VSS  G$9:AV23.VSS  out
AV24.CLK_REQ1_L/AGPIO115  G$10:AV24.CLK_REQ1_L/AGPIO115
AV25.SDA0/I2C2_SDA/EGPIO114  G$10:AV25.SDA0/I2C2_SDA/EGPIO114
AV26.VSS  G$9:AV26.VSS  out
AV27.MB_DATA[63]  G$2:AV27.MB_DATA[63]
AV28.MB_DATA[62]  G$2:AV28.MB_DATA[62]
AV29.VSS  G$9:AV29.VSS  out
AV30.MB_DATA[57]  G$2:AV30.MB_DATA[57]
AV31.MB_DATA[60]  G$2:AV31.MB_DATA[60]
AV32.VSS  G$9:AV32.VSS  out
AV33.MB_DATA[55]  G$2:AV33.MB_DATA[55]
AV34.MB_DQS_L[6]  G$2:AV34.MB_DQS_L[6]
AV35.VSS  G$9:AV35.VSS  out
AV36.MB_DATA[52]  G$2:AV36.MB_DATA[52]
AV37.MB_DATA[43]  G$2:AV37.MB_DATA[43]
AV38.VSS  G$9:AV38.VSS  out
AW3.AZ_BITCLK  G$10:AW3.AZ_BITCLK
AW4.VSS  G$9:AW4.VSS  out
AW5.X32K_X1  G$10:AW5.X32K_X1
AW6.X32K_X2  G$10:AW6.X32K_X2
AW7.VSS  G$9:AW7.VSS  out
AW8.USB_HSD1P  G$4:AW8.USB_HSD1P
AW9.USB_HSD1N  G$4:AW9.USB_HSD1N
AW10.VSS  G$9:AW10.VSS  out
AW11.EGPIO95  G$10:AW11.EGPIO95
AW12.EGPIO97  G$10:AW12.EGPIO97
AW13.VSS  G$9:AW13.VSS  out
AW14.SPI_CLK/ESPI_CLK/EGPIO117  G$4:AW14.SPI_CLK/ESPI_CLK/EGPIO117
AW15.SPI_CS2_L/ESPI_CS_L/EGPIO119  G$4:AW15.SPI_CS2_L/ESPI_CS_L/EGPIO119
AW16.VSS  G$9:AW16.VSS  out
AW17.AGPIO86  G$10:AW17.AGPIO86
AW18.LFRAME_L/EGPIO109  G$4:AW18.LFRAME_L/EGPIO109
AW19.VSS  G$9:AW19.VSS  out
AW20.LAD0/EGPIO104  G$4:AW20.LAD0/EGPIO104
AW21.SERIRQ/AGPIO87  G$4:AW21.SERIRQ/AGPIO87
AW22.VSS  G$9:AW22.VSS  out
AW23.SPKR/AGPIO91  G$10:AW23.SPKR/AGPIO91
AW24.RSVD  G$7:AW24.RSVD  nc
AW25.VSS  G$9:AW25.VSS  out
AW26.MB_DATA[59]  G$2:AW26.MB_DATA[59]
AW27.MB_DATA[58]  G$2:AW27.MB_DATA[58]
AW28.VSS  G$9:AW28.VSS  out
AW29.MB_DM[7]  G$2:AW29.MB_DM[7]
AW30.MB_DATA[56]  G$2:AW30.MB_DATA[56]
AW31.VSS  G$9:AW31.VSS  out
AW32.MB_DATA[50]  G$2:AW32.MB_DATA[50]
AW33.MB_DATA[54]  G$2:AW33.MB_DATA[54]
AW34.VSS  G$9:AW34.VSS  out
AW35.MB_DATA[48]  G$2:AW35.MB_DATA[48]
AW36.MB_DATA[53]  G$2:AW36.MB_DATA[53]
AW37.VSS  G$9:AW37.VSS  out
B3.DP0_TXN[1]  G$3:B3.DP0_TXN[1]
B4.DP0_TXP[2]  G$3:B4.DP0_TXP[2]
B5.VDDCR_SOC  G$6:B5.VDDCR_SOC  pwr
B6.DP2_TXP[0]  G$3:B6.DP2_TXP[0]
B7.DP2_TXN[0]  G$3:B7.DP2_TXN[0]
B8.VDDCR_SOC  G$6:B8.VDDCR_SOC  pwr
B9.DP2_TXP[3]  G$3:B9.DP2_TXP[3]
B10.DP2_TXN[3]  G$3:B10.DP2_TXN[3]
B11.VDDCR_SOC  G$6:B11.VDDCR_SOC  pwr
B12.TEST15  G$3:B12.TEST15
B13.TRST_L  G$3:B13.TRST_L
B14.VDDCR_SOC  G$6:B14.VDDCR_SOC  pwr
B15.TMS  G$3:B15.TMS
B16.RESET_L  G$3:B16.RESET_L
B17.VDDCR_SOC  G$6:B17.VDDCR_SOC  pwr
B18.SIC  G$3:B18.SIC
B19.VSS  G$9:B19.VSS  out
B20.VDDCR_SOC  G$6:B20.VDDCR_SOC  pwr
B21.MB_DATA[1]  G$2:B21.MB_DATA[1]
B22.MB_DQS_H[0]  G$2:B22.MB_DQS_H[0]
B23.VSS  G$9:B23.VSS  out
B24.MB_DATA[2]  G$2:B24.MB_DATA[2]
B25.MB_DATA[13]  G$2:B25.MB_DATA[13]
B26.VSS  G$9:B26.VSS  out
B27.MB_DQS_L[1]  G$2:B27.MB_DQS_L[1]
B28.MB_DATA[15]  G$2:B28.MB_DATA[15]
B29.VSS  G$9:B29.VSS  out
B30.MB_DATA[20]  G$2:B30.MB_DATA[20]
B31.MB_DATA[17]  G$2:B31.MB_DATA[17]
B32.VSS  G$9:B32.VSS  out
B33.MB_DATA[22]  G$2:B33.MB_DATA[22]
B34.MB_DATA[18]  G$2:B34.MB_DATA[18]
B35.VSS  G$9:B35.VSS  out
B36.MB_DATA[24]  G$2:B36.MB_DATA[24]
B37.MB_DQS_H[3]  G$2:B37.MB_DQS_H[3]
B38.MB_DATA[30]  G$2:B38.MB_DATA[30]
C1.VSS  G$9:C1.VSS  out
C2.DP0_TXN[0]  G$3:C2.DP0_TXN[0]
C3.DP0_TXP[1]  G$3:C3.DP0_TXP[1]
C4.VDDCR_SOC  G$6:C4.VDDCR_SOC  pwr
C5.DP0_TXP[3]  G$3:C5.DP0_TXP[3]
C6.DP0_TXN[3]  G$3:C6.DP0_TXN[3]
C7.VDDCR_SOC  G$6:C7.VDDCR_SOC  pwr
C8.DP2_TXP[2]  G$3:C8.DP2_TXP[2]
C9.DP2_TXN[2]  G$3:C9.DP2_TXN[2]
C10.VDDCR_SOC  G$6:C10.VDDCR_SOC  pwr
C11.TEST16  G$3:C11.TEST16
C12.TEST14  G$3:C12.TEST14
C13.VDDCR_SOC  G$6:C13.VDDCR_SOC  pwr
C14.TDO  G$3:C14.TDO
C15.TCK  G$3:C15.TCK
C16.VDDCR_SOC  G$6:C16.VDDCR_SOC  pwr
C17.SVD  G$3:C17.SVD
C18.SID  G$3:C18.SID
C19.VDDCR_SOC  G$6:C19.VDDCR_SOC  pwr
C20.MB_DATA[5]  G$2:C20.MB_DATA[5]
C21.MB_DM[0]  G$2:C21.MB_DM[0]
C22.VSS  G$9:C22.VSS  out
C23.MB_DATA[7]  G$2:C23.MB_DATA[7]
C24.MB_DATA[3]  G$2:C24.MB_DATA[3]
C25.VSS  G$9:C25.VSS  out
C26.MB_DATA[9]  G$2:C26.MB_DATA[9]
C27.MB_DQS_H[1]  G$2:C27.MB_DQS_H[1]
C28.VSS  G$9:C28.VSS  out
C29.MB_DATA[11]  G$2:C29.MB_DATA[11]
C30.MB_DATA[21]  G$2:C30.MB_DATA[21]
C31.VSS  G$9:C31.VSS  out
C32.MB_DQS_L[2]  G$2:C32.MB_DQS_L[2]
C33.MB_DQS_H[2]  G$2:C33.MB_DQS_H[2]
C34.VSS  G$9:C34.VSS  out
C35.MB_DATA[19]  G$2:C35.MB_DATA[19]
C36.MB_DATA[29]  G$2:C36.MB_DATA[29]
C37.VSS  G$9:C37.VSS  out
C38.MB_DATA[31]  G$2:C38.MB_DATA[31]
C39.MB_DATA[26]  G$2:C39.MB_DATA[26]
D1.P_GFX_TXP[0]  G$5:D1.P_GFX_TXP[0]
D2.DP0_TXP[0]  G$3:D2.DP0_TXP[0]
D3.VDDCR_SOC  G$6:D3.VDDCR_SOC  pwr
D4.DP1_TXP[0]  G$3:D4.DP1_TXP[0]
D5.DP1_TXN[0]  G$3:D5.DP1_TXN[0]
D6.VSS  G$9:D6.VSS  out
D7.DP1_TXP[1]  G$3:D7.DP1_TXP[1]
D8.DP1_TXN[1]  G$3:D8.DP1_TXN[1]
D9.VSS  G$9:D9.VSS  out
D10.DP1_HPD  G$3:D10.DP1_HPD
D11.TEST17  G$3:D11.TEST17
D12.VSS  G$9:D12.VSS  out
D13.TEST6  G$3:D13.TEST6
D14.DBREQ_L  G$3:D14.DBREQ_L
D15.VSS  G$9:D15.VSS  out
D16.ALERT_L  G$3:D16.ALERT_L
D17.SVC  G$3:D17.SVC
D18.VSS  G$9:D18.VSS  out
D19.VSS  G$9:D19.VSS  out
D20.MB_DATA[0]  G$2:D20.MB_DATA[0]
D21.VSS  G$9:D21.VSS  out
D22.VSS  G$9:D22.VSS  out
D23.VSS  G$9:D23.VSS  out
D24.VSS  G$9:D24.VSS  out
D25.VSS  G$9:D25.VSS  out
D26.MB_DM[1]  G$2:D26.MB_DM[1]
D27.VSS  G$9:D27.VSS  out
D28.RSVD  G$7:D28.RSVD  nc
D29.VSS  G$9:D29.VSS  out
D30.VSS  G$9:D30.VSS  out
D31.VSS  G$9:D31.VSS  out
D32.VSS  G$9:D32.VSS  out
D33.VSS  G$9:D33.VSS  out
D34.VSS  G$9:D34.VSS  out
D35.VSS  G$9:D35.VSS  out
D36.VSS  G$9:D36.VSS  out
D37.MB_DM[3]  G$2:D37.MB_DM[3]
D38.MB_DATA[27]  G$2:D38.MB_DATA[27]
D39.VSS  G$9:D39.VSS  out
E1.P_GFX_TXN[0]  G$5:E1.P_GFX_TXN[0]
E2.VDDCR_SOC  G$6:E2.VDDCR_SOC  pwr
E3.P_GFX_TXP[1]  G$5:E3.P_GFX_TXP[1]
E4.VSS  G$9:E4.VSS  out
E5.VSS  G$9:E5.VSS  out
E6.TEST28_H  G$3:E6.TEST28_H
E7.TEST28_L  G$3:E7.TEST28_L
E8.VSS  G$9:E8.VSS  out
E9.DP1_TXP[3]  G$3:E9.DP1_TXP[3]
E10.DP2_HPD  G$3:E10.DP2_HPD
E11.VSS  G$9:E11.VSS  out
E12.DP_AUX_ZVSS  G$3:E12.DP_AUX_ZVSS  out
E13.DBRDY  G$3:E13.DBRDY
E14.VSS  G$9:E14.VSS  out
E15.VDDCR_SOC_SENSE  G$3:E15.VDDCR_SOC_SENSE  pwr
E16.PWROK  G$3:E16.PWROK
E17.VSS  G$9:E17.VSS  out
E18.MA_DATA[0]  G$1:E18.MA_DATA[0]
E19.RSVD  G$7:E19.RSVD  nc
E20.VSS  G$9:E20.VSS  out
E21.VSS  G$9:E21.VSS  out
E22.RSVD  G$7:E22.RSVD  nc
E23.VSS  G$9:E23.VSS  out
E24.MA_DATA[10]  G$1:E24.MA_DATA[10]
E25.RSVD  G$7:E25.RSVD  nc
E26.VSS  G$9:E26.VSS  out
E27.VSS  G$9:E27.VSS  out
E28.MA_DATA[22]  G$1:E28.MA_DATA[22]
E29.VSS  G$9:E29.VSS  out
E30.MA_DQS_L[3]  G$1:E30.MA_DQS_L[3]
E31.MA_DATA[30]  G$1:E31.MA_DATA[30]
E32.VSS  G$9:E32.VSS  out
E33.MA_CHECK[4]  G$1:E33.MA_CHECK[4]
E34.MA_CHECK[5]  G$1:E34.MA_CHECK[5]
E35.VSS  G$9:E35.VSS  out
E36.MB_DATA[25]  G$2:E36.MB_DATA[25]
E37.MB_CHECK[4]  G$2:E37.MB_CHECK[4]
E38.VSS  G$9:E38.VSS  out
E39.MB_CHECK[5]  G$2:E39.MB_CHECK[5]
F1.VSS  G$9:F1.VSS  out
F2.P_GFX_TXP[2]  G$5:F2.P_GFX_TXP[2]
F3.P_GFX_TXN[1]  G$5:F3.P_GFX_TXN[1]
F4.VSS  G$9:F4.VSS  out
F5.P_GFX_RXN[0]  G$5:F5.P_GFX_RXN[0]
F6.P_GFX_RXP[0]  G$5:F6.P_GFX_RXP[0]
F7.VDDCR_SOC  G$6:F7.VDDCR_SOC  pwr
F8.DP1_TXP[2]  G$3:F8.DP1_TXP[2]
F9.DP1_TXN[3]  G$3:F9.DP1_TXN[3]
F10.VDDCR_SOC  G$6:F10.VDDCR_SOC  pwr
F11.DP1_AUXP  G$3:F11.DP1_AUXP
F12.DP_ZVSS  G$3:F12.DP_ZVSS  out
F13.VDDCR_SOC  G$6:F13.VDDCR_SOC  pwr
F14.VDDCR_CPU_SENSE  G$3:F14.VDDCR_CPU_SENSE  pwr
F15.VSS_SENSE_A  G$3:F15.VSS_SENSE_A
F16.VDDCR_SOC  G$6:F16.VDDCR_SOC  pwr
F17.VSS  G$9:F17.VSS  out
F18.MA_DATA[5]  G$1:F18.MA_DATA[5]
F19.VSS  G$9:F19.VSS  out
F20.MA_DATA[7]  G$1:F20.MA_DATA[7]
F21.MA_DATA[12]  G$1:F21.MA_DATA[12]
F22.VSS  G$9:F22.VSS  out
F23.MA_DQS_H[1]  G$1:F23.MA_DQS_H[1]
F24.MA_DATA[15]  G$1:F24.MA_DATA[15]
F25.VSS  G$9:F25.VSS  out
F26.MA_DQS_L[2]  G$1:F26.MA_DQS_L[2]
F27.MA_DQS_H[2]  G$1:F27.MA_DQS_H[2]
F28.VSS  G$9:F28.VSS  out
F29.MA_DATA[24]  G$1:F29.MA_DATA[24]
F30.MA_DQS_H[3]  G$1:F30.MA_DQS_H[3]
F31.VSS  G$9:F31.VSS  out
F32.MA_DATA[27]  G$1:F32.MA_DATA[27]
F33.MA_CHECK[0]  G$1:F33.MA_CHECK[0]
F34.VSS  G$9:F34.VSS  out
F35.VSS  G$9:F35.VSS  out
F36.MB_CHECK[1]  G$2:F36.MB_CHECK[1]
F37.VSS  G$9:F37.VSS  out
F38.MB_CHECK[0]  G$2:F38.MB_CHECK[0]
F39.MB_DM[8]  G$2:F39.MB_DM[8]
G1.P_GFX_TXP[3]  G$5:G1.P_GFX_TXP[3]
G2.P_GFX_TXN[2]  G$5:G2.P_GFX_TXN[2]
G3.VDDCR_SOC  G$6:G3.VDDCR_SOC  pwr
G4.P_GFX_RXN[1]  G$5:G4.P_GFX_RXN[1]
G5.P_GFX_RXP[1]  G$5:G5.P_GFX_RXP[1]
G6.VDDCR_SOC  G$6:G6.VDDCR_SOC  pwr
G7.VSS  G$9:G7.VSS  out
G8.DP1_TXN[2]  G$3:G8.DP1_TXN[2]
G9.VDDCR_SOC  G$6:G9.VDDCR_SOC  pwr
G10.DP0_AUXP  G$3:G10.DP0_AUXP
G11.DP1_AUXN  G$3:G11.DP1_AUXN
G12.VDDCR_SOC  G$6:G12.VDDCR_SOC  pwr
G13.DP_BLON  G$3:G13.DP_BLON
G14.VDDIO_MEM_S3_SENSE  G$3:G14.VDDIO_MEM_S3_SENSE  pwr
G15.VDDCR_SOC  G$6:G15.VDDCR_SOC  pwr
G16.TEST18  G$3:G16.TEST18
G17.RSVD  G$7:G17.RSVD  nc
G18.VDDCR_SOC  G$6:G18.VDDCR_SOC  pwr
G19.MA_DQS_L[0]  G$1:G19.MA_DQS_L[0]
G20.MA_DATA[6]  G$1:G20.MA_DATA[6]
G21.VSS  G$9:G21.VSS  out
G22.MA_DATA[9]  G$1:G22.MA_DATA[9]
G23.MA_DQS_L[1]  G$1:G23.MA_DQS_L[1]
G24.VSS  G$9:G24.VSS  out
G25.MA_DATA[21]  G$1:G25.MA_DATA[21]
G26.MA_DM[2]  G$1:G26.MA_DM[2]
G27.VSS  G$9:G27.VSS  out
G28.MA_DATA[18]  G$1:G28.MA_DATA[18]
G29.MA_DATA[29]  G$1:G29.MA_DATA[29]
G30.VSS  G$9:G30.VSS  out
G31.MA_DATA[31]  G$1:G31.MA_DATA[31]
G32.MA_CHECK[1]  G$1:G32.MA_CHECK[1]
G33.VSS  G$9:G33.VSS  out
G34.MA_DM[8]  G$1:G34.MA_DM[8]
G35.VSS  G$9:G35.VSS  out
G36.VSS  G$9:G36.VSS  out
G37.MB_DQS_L[8]  G$2:G37.MB_DQS_L[8]
G38.MB_DQS_H[8]  G$2:G38.MB_DQS_H[8]
G39.VSS  G$9:G39.VSS  out
H1.P_GFX_TXN[3]  G$5:H1.P_GFX_TXN[3]
H2.VDDCR_SOC  G$6:H2.VDDCR_SOC  pwr
H3.P_GFX_TXP[4]  G$5:H3.P_GFX_TXP[4]
H4.VSS  G$9:H4.VSS  out
H5.VSS  G$9:H5.VSS  out
H6.P_GFX_RXN[2]  G$5:H6.P_GFX_RXN[2]
H7.P_GFX_RXP[2]  G$5:H7.P_GFX_RXP[2]
H8.VSS  G$9:H8.VSS  out
H9.DP0_HPD  G$3:H9.DP0_HPD
H10.DP0_AUXN  G$3:H10.DP0_AUXN
H11.VSS  G$9:H11.VSS  out
H12.DP_VARYBL  G$3:H12.DP_VARYBL
H13.DP_DIGON  G$3:H13.DP_DIGON
H14.VSS  G$9:H14.VSS  out
H15.PROCHOT_L  G$3:H15.PROCHOT_L
H16.TEST19  G$3:H16.TEST19
H17.VSS  G$9:H17.VSS  out
H18.MA_DATA[4]  G$1:H18.MA_DATA[4]
H19.MA_DQS_H[0]  G$1:H19.MA_DQS_H[0]
H20.VSS  G$9:H20.VSS  out
H21.MA_DATA[3]  G$1:H21.MA_DATA[3]
H22.MA_DATA[8]  G$1:H22.MA_DATA[8]
H23.VSS  G$9:H23.VSS  out
H24.MA_DATA[14]  G$1:H24.MA_DATA[14]
H25.MA_DATA[20]  G$1:H25.MA_DATA[20]
H26.VSS  G$9:H26.VSS  out
H27.MA_DATA[23]  G$1:H27.MA_DATA[23]
H28.MA_DATA[19]  G$1:H28.MA_DATA[19]
H29.VSS  G$9:H29.VSS  out
H30.MA_DM[3]  G$1:H30.MA_DM[3]
H31.MA_DATA[26]  G$1:H31.MA_DATA[26]
H32.VSS  G$9:H32.VSS  out
H33.MA_DQS_L[8]  G$1:H33.MA_DQS_L[8]
H34.MA_DQS_H[8]  G$1:H34.MA_DQS_H[8]
H35.VSS  G$9:H35.VSS  out
H36.MB_CHECK[6]  G$2:H36.MB_CHECK[6]
H37.MB_CHECK[7]  G$2:H37.MB_CHECK[7]
H38.VSS  G$9:H38.VSS  out
H39.MB_CHECK[2]  G$2:H39.MB_CHECK[2]
J1.VSS  G$9:J1.VSS  out
J2.P-GFX_TXP[5]  G$5:J2.P-GFX_TXP[5]
J3.P_GFX_TXN[4]  G$5:J3.P_GFX_TXN[4]
J4.VSS  G$9:J4.VSS  out
J5.P_GFX_RXN[3]  G$5:J5.P_GFX_RXN[3]
J6.P_GFX_RXP[3]  G$5:J6.P_GFX_RXP[3]
J7.VDDCR_SOC  G$6:J7.VDDCR_SOC  pwr
J8.VSS  G$9:J8.VSS  out
J9.VSS  G$9:J9.VSS  out
J10.VDDCR_SOC  G$6:J10.VDDCR_SOC  pwr
J11.VSS  G$9:J11.VSS  out
J12.VDDCR_SOC  G$6:J12.VDDCR_SOC  pwr
J13.VSS  G$9:J13.VSS  out
J14.VDDCR_SOC  G$6:J14.VDDCR_SOC  pwr
J15.VSS  G$9:J15.VSS  out
J16.VDDCR_SOC  G$6:J16.VDDCR_SOC  pwr
J17.VSS  G$9:J17.VSS  out
J18.MA_DATA[1]  G$1:J18.MA_DATA[1]
J19.VSS  G$9:J19.VSS  out
J20.MA_DATA[2]  G$1:J20.MA_DATA[2]
J21.MA_DATA[13]  G$1:J21.MA_DATA[13]
J22.VSS  G$9:J22.VSS  out
J23.MA_DM[1]  G$1:J23.MA_DM[1]
J24.MA_DATA[11]  G$1:J24.MA_DATA[11]
J25.VSS  G$9:J25.VSS  out
J26.MA_DATA[16]  G$1:J26.MA_DATA[16]
J27.MA_DATA[17]  G$1:J27.MA_DATA[17]
J28.VSS  G$9:J28.VSS  out
J29.MA_DATA[28]  G$1:J29.MA_DATA[28]
J30.MA_DATA[25]  G$1:J30.MA_DATA[25]
J31.VSS  G$9:J31.VSS  out
J32.MA_CHECK[6]  G$1:J32.MA_CHECK[6]
J33.MA_CHECK[7]  G$1:J33.MA_CHECK[7]
J34.VSS  G$9:J34.VSS  out
J35.VSS  G$9:J35.VSS  out
J36.RSVD  G$7:J36.RSVD  nc
J37.VSS  G$9:J37.VSS  out
J38.RSVD  G$7:J38.RSVD  nc
J39.MB_CHECK[3]  G$2:J39.MB_CHECK[3]
K1.P_GFX_TXP[6]  G$5:K1.P_GFX_TXP[6]
K2.P_GFX_TXN[5]  G$5:K2.P_GFX_TXN[5]
K3.VDDCR_SOC  G$6:K3.VDDCR_SOC  pwr
K4.P_GFX_RXN[5]  G$5:K4.P_GFX_RXN[5]
K5.P_GFX_RXP[5]  G$5:K5.P_GFX_RXP[5]
K6.VDDCR_SOC  G$6:K6.VDDCR_SOC  pwr
K7.P_GFX_RXN[4]  G$5:K7.P_GFX_RXN[4]
K8.P_GFX_RXP[4]  G$5:K8.P_GFX_RXP[4]
K9.VDDCR_SOC  G$6:K9.VDDCR_SOC  pwr
K10.VSS  G$9:K10.VSS  out
K11.VDDCR_SOC  G$6:K11.VDDCR_SOC  pwr
K12.VSS  G$9:K12.VSS  out
K13.VDDCR_SOC  G$6:K13.VDDCR_SOC  pwr
K14.DP_STEREOSYNC  G$3:K14.DP_STEREOSYNC
K15.VDDCR_SOC  G$6:K15.VDDCR_SOC  pwr
K18.VSS  G$9:K18.VSS  out
K19.MA_DM[0]  G$1:K19.MA_DM[0]
K20.VSS  G$9:K20.VSS  out
K21.VSS  G$9:K21.VSS  out
K22.VSS  G$9:K22.VSS  out
K23.VSS  G$9:K23.VSS  out
K26.VSS  G$9:K26.VSS  out
K27.VSS  G$9:K27.VSS  out
K28.VSS  G$9:K28.VSS  out
K29.VSS  G$9:K29.VSS  out
K30.VSS  G$9:K30.VSS  out
K31.MA_CHECK[2]  G$1:K31.MA_CHECK[2]
K32.MA_CHECK[3]  G$1:K32.MA_CHECK[3]
K33.VSS  G$9:K33.VSS  out
K34.RSVD  G$7:K34.RSVD  nc
K35.MB_RESET_L  G$2:K35.MB_RESET_L
K36.VDDIO_MEM_S3  G$8:K36.VDDIO_MEM_S3  pwr
K37.MB0_CKE[1]  G$2:K37.MB0_CKE[1]
K38.RSVD  G$7:K38.RSVD  nc
K39.VDDIO_MEM_S3  G$8:K39.VDDIO_MEM_S3  pwr
L1.P_GFX_TXN[6]  G$5:L1.P_GFX_TXN[6]
L2.VDDCR_SOC  G$6:L2.VDDCR_SOC  pwr
L3.P_GFX_TXP[7]  G$5:L3.P_GFX_TXP[7]
L4.VSS  G$9:L4.VSS  out
L5.VSS  G$9:L5.VSS  out
L6.P_GFX_RXN[6]  G$5:L6.P_GFX_RXN[6]
L7.P_GFX_RXP[6]  G$5:L7.P_GFX_RXP[6]
L8.VSS  G$9:L8.VSS  out
L9.VSS  G$9:L9.VSS  out
L10.VDDCR_SOC  G$6:L10.VDDCR_SOC  pwr
L11.VSS  G$9:L11.VSS  out
L12.VDDCR_SOC  G$6:L12.VDDCR_SOC  pwr
L13.VSS  G$9:L13.VSS  out
L14.VDDCR_SOC  G$6:L14.VDDCR_SOC  pwr
L15.VSS  G$9:L15.VSS  out
L16.VDDCR_SOC  G$6:L16.VDDCR_SOC  pwr
L17.VSS  G$9:L17.VSS  out
L18.VDDCR_SOC  G$6:L18.VDDCR_SOC  pwr
L19.VSS  G$9:L19.VSS  out
L20.VDDCR_SOC  G$6:L20.VDDCR_SOC  pwr
L21.VSS  G$9:L21.VSS  out
L22.VDDCR_SOC  G$6:L22.VDDCR_SOC  pwr
L23.TEST4  G$3:L23.TEST4
L24.VDDCR_SOC  G$6:L24.VDDCR_SOC  pwr
L25.VSS  G$9:L25.VSS  out
L26.VDDCR_SOC  G$6:L26.VDDCR_SOC  pwr
L27.VSS  G$9:L27.VSS  out
L28.VSS  G$9:L28.VSS  out
L29.VSS  G$9:L29.VSS  out
L30.VSS  G$9:L30.VSS  out
L31.VSS  G$9:L31.VSS  out
L32.VDDIO_MEM_S3  G$8:L32.VDDIO_MEM_S3  pwr
L33.MA_RESET_L  G$1:L33.MA_RESET_L
L34.MA1_CKE[1]  G$1:L34.MA1_CKE[1]
L35.VDDIO_MEM_S3  G$8:L35.VDDIO_MEM_S3  pwr
L36.MB1_CKE[1]  G$2:L36.MB1_CKE[1]
L37.MB0_CKE[0]  G$2:L37.MB0_CKE[0]
L38.VDDIO_MEM_S3  G$8:L38.VDDIO_MEM_S3  pwr
L39.MB1_CKE[0]  G$2:L39.MB1_CKE[0]
M1.VSS  G$9:M1.VSS  out
M2.P_GFX_TXP[8]  G$5:M2.P_GFX_TXP[8]
M3.P_GFX_TXN[7]  G$5:M3.P_GFX_TXN[7]
M4.VSS  G$9:M4.VSS  out
M5.P_GFX_RXN[7]  G$5:M5.P_GFX_RXN[7]
M6.P_GFX_RXP[7]  G$5:M6.P_GFX_RXP[7]
M7.VDDCR_CPU  G$6:M7.VDDCR_CPU  pwr
M8.VSS  G$9:M8.VSS  out
M9.VDDCR_SOC  G$6:M9.VDDCR_SOC  pwr
M10.VSS  G$9:M10.VSS  out
M11.VDDCR_SOC  G$6:M11.VDDCR_SOC  pwr
M12.VSS  G$9:M12.VSS  out
M13.VDDCR_SOC  G$6:M13.VDDCR_SOC  pwr
M14.VSS  G$9:M14.VSS  out
M15.VDDCR_SOC  G$6:M15.VDDCR_SOC  pwr
M16.VSS  G$9:M16.VSS  out
M17.VDDCR_SOC  G$6:M17.VDDCR_SOC  pwr
M18.VSS  G$9:M18.VSS  out
M19.VDDCR_SOC  G$6:M19.VDDCR_SOC  pwr
M20.VSS  G$9:M20.VSS  out
M21.VDDCR_SOC  G$6:M21.VDDCR_SOC  pwr
M22.TEST5  G$3:M22.TEST5
M23.VDDCR_SOC  G$6:M23.VDDCR_SOC  pwr
M24.VSS  G$9:M24.VSS  out
M25.VDDCR_SOC  G$6:M25.VDDCR_SOC  pwr
M26.VSS  G$9:M26.VSS  out
M27.VSS  G$9:M27.VSS  out
M28.VSS  G$9:M28.VSS  out
M29.VDDIO_MEM_S3  G$8:M29.VDDIO_MEM_S3  pwr
M30.MA0_CKE[1]  G$1:M30.MA0_CKE[1]
M31.VDDIO_MEM_S3  G$8:M31.VDDIO_MEM_S3  pwr
M32.MA0_CKE[0]  G$1:M32.MA0_CKE[0]
M33.MA1_CKE[0]  G$1:M33.MA1_CKE[0]
M34.VDDIO_MEM_S3  G$8:M34.VDDIO_MEM_S3  pwr
M35.MA_ACT_L  G$1:M35.MA_ACT_L
M36.MB_BG[0]  G$2:M36.MB_BG[0]
M37.VDDIO_MEM_S3  G$8:M37.VDDIO_MEM_S3  pwr
M38.MB_ACT_L  G$2:M38.MB_ACT_L
M39.MB_BG[1]  G$2:M39.MB_BG[1]
N1.P_GFX_TXP[9]  G$5:N1.P_GFX_TXP[9]
N2.P_GFX_TXN[8]  G$5:N2.P_GFX_TXN[8]
N3.VDDCR_CPU  G$6:N3.VDDCR_CPU  pwr
N4.P_GFX_RXN[9]  G$5:N4.P_GFX_RXN[9]
N5.P_GFX_RXP[9]  G$5:N5.P_GFX_RXP[9]
N6.VDDCR_CPU  G$6:N6.VDDCR_CPU  pwr
N7.P_GFX_RXN[8]  G$5:N7.P_GFX_RXN[8]
N8.P_GFX_RXP[8]  G$5:N8.P_GFX_RXP[8]
N9.VSS  G$9:N9.VSS  out
N10.VDDCR_SOC  G$6:N10.VDDCR_SOC  pwr
N11.VSS  G$9:N11.VSS  out
N12.VDDCR_SOC  G$6:N12.VDDCR_SOC  pwr
N13.VSS  G$9:N13.VSS  out
N14.VDDCR_SOC  G$6:N14.VDDCR_SOC  pwr
N15.VSS  G$9:N15.VSS  out
N16.VDDCR_SOC  G$6:N16.VDDCR_SOC  pwr
N17.VSS  G$9:N17.VSS  out
N18.VDDCR_SOC  G$6:N18.VDDCR_SOC  pwr
N19.VSS  G$9:N19.VSS  out
N20.VDDCR_SOC  G$6:N20.VDDCR_SOC  pwr
N21.VSS  G$9:N21.VSS  out
N22.VDDCR_SOC  G$6:N22.VDDCR_SOC  pwr
N23.VSS  G$9:N23.VSS  out
N24.VDDCR_SOC  G$6:N24.VDDCR_SOC  pwr
N25.VSS  G$9:N25.VSS  out
N26.VDDCR_SOC  G$6:N26.VDDCR_SOC  pwr
N27.VSS  G$9:N27.VSS  out
N28.VDDIO_MEM_S3  G$8:N28.VDDIO_MEM_S3  pwr
N29.VSS  G$9:N29.VSS  out
N30.VDDIO_MEM_S3  G$8:N30.VDDIO_MEM_S3  pwr
N31.MA_BG[0]  G$1:N31.MA_BG[0]
N32.MA_BG[1]  G$1:N32.MA_BG[1]
N33.VDDIO_MEM_S3  G$8:N33.VDDIO_MEM_S3  pwr
N34.MA_ALERT_L  G$1:N34.MA_ALERT_L
N35.MA_ADD[12]  G$1:N35.MA_ADD[12]
N36.VDDIO_MEM_S3  G$8:N36.VDDIO_MEM_S3  pwr
N37.MB_ALERT_L  G$2:N37.MB_ALERT_L
N38.MB_ADD[12]  G$2:N38.MB_ADD[12]
N39.VDDIO_MEM_S3  G$8:N39.VDDIO_MEM_S3  pwr
P1.P_GFX_TXN[9]  G$5:P1.P_GFX_TXN[9]
P2.VDDCR_CPU  G$6:P2.VDDCR_CPU  pwr
P3.P_GFX_TXP[10]  G$5:P3.P_GFX_TXP[10]
P4.VSS  G$9:P4.VSS  out
P5.VSS  G$9:P5.VSS  out
P6.P_GFX_RXN[10]  G$5:P6.P_GFX_RXN[10]
P7.P_GFX_RXP[10]  G$5:P7.P_GFX_RXP[10]
P8.VSS  G$9:P8.VSS  out
P9.VDDCR_SOC  G$6:P9.VDDCR_SOC  pwr
P10.VSS  G$9:P10.VSS  out
P11.VDDCR_SOC  G$6:P11.VDDCR_SOC  pwr
P12.VSS  G$9:P12.VSS  out
P13.VDDCR_SOC  G$6:P13.VDDCR_SOC  pwr
P27.VDDIO_MEM_S3  G$8:P27.VDDIO_MEM_S3  pwr
P28.TEST47  G$3:P28.TEST47
P29.VDDIO_MEM_S3  G$8:P29.VDDIO_MEM_S3  pwr
P30.MA_ADD[8]  G$1:P30.MA_ADD[8]
P31.MA_ADD[9]  G$1:P31.MA_ADD[9]
P32.VDDIO_MEM_S3  G$8:P32.VDDIO_MEM_S3  pwr
P33.MA_ADD[11]  G$1:P33.MA_ADD[11]
P34.MA_ADD[7]  G$1:P34.MA_ADD[7]
P35.VDDIO_MEM_S3  G$8:P35.VDDIO_MEM_S3  pwr
P36.MB_ADD[9]  G$2:P36.MB_ADD[9]
P37.MB_ADD[11]  G$2:P37.MB_ADD[11]
P38.VDDIO_MEM_S3  G$8:P38.VDDIO_MEM_S3  pwr
P39.MB_ADD[7]  G$2:P39.MB_ADD[7]
R1.VSS  G$9:R1.VSS  out
R2.P_GFX_TXP[11]  G$5:R2.P_GFX_TXP[11]
R3.P_GFX_TXN[10]  G$5:R3.P_GFX_TXN[10]
R4.VSS  G$9:R4.VSS  out
R5.P_GFX_RXN[11]  G$5:R5.P_GFX_RXN[11]
R6.P_GFX_RXP[11]  G$5:R6.P_GFX_RXP[11]
R7.VDDCR_CPU  G$6:R7.VDDCR_CPU  pwr
R8.VSS  G$9:R8.VSS  out
R9.VSS  G$9:R9.VSS  out
R10.VDDCR-SOC  G$6:R10.VDDCR-SOC  pwr
R11.VSS  G$9:R11.VSS  out
R12.VDDCR_SOC  G$6:R12.VDDCR_SOC  pwr
R13.VSS  G$9:R13.VSS  out
R27.VSS  G$9:R27.VSS  out
R28.VDDIO_MEM_S3  G$8:R28.VDDIO_MEM_S3  pwr
R29.VSS  G$9:R29.VSS  out
R30.MA_ADD[4]  G$1:R30.MA_ADD[4]
R31.VDDIO_MEM_S3  G$8:R31.VDDIO_MEM_S3  pwr
R32.MA_ADD[6]  G$1:R32.MA_ADD[6]
R33.MA_ADD[5]  G$1:R33.MA_ADD[5]
R34.VDDIO_MEM_S3  G$8:R34.VDDIO_MEM_S3  pwr
R35.RSVD  G$7:R35.RSVD  nc
R36.MB_ADD[6]  G$2:R36.MB_ADD[6]
R37.VDDIO_MEM_S3  G$8:R37.VDDIO_MEM_S3  pwr
R38.MB_ADD[8]  G$2:R38.MB_ADD[8]
R39.MB_ADD[5]  G$2:R39.MB_ADD[5]
T1.P_GFX_TXP[12]  G$5:T1.P_GFX_TXP[12]
T2.P_GFX_TXN[11]  G$5:T2.P_GFX_TXN[11]
T3.VDDCR_CPU  G$6:T3.VDDCR_CPU  pwr
T4.P_GFX_RXP[13]  G$5:T4.P_GFX_RXP[13]
T5.P_GFX_RXN[13]  G$5:T5.P_GFX_RXN[13]
T6.VDDCR_CPU  G$6:T6.VDDCR_CPU  pwr
T7.P_GFX_RXN[12]  G$5:T7.P_GFX_RXN[12]
T8.P_GFX_RXP[12]  G$5:T8.P_GFX_RXP[12]
T9.VDDCR_CPU  G$6:T9.VDDCR_CPU  pwr
T10.VSS  G$9:T10.VSS  out
T11.VDDCR_SOC  G$6:T11.VDDCR_SOC  pwr
T12.VSS  G$9:T12.VSS  out
T13.VDDCR_SOC  G$6:T13.VDDCR_SOC  pwr
T27.VDDIO_MEM_S3  G$8:T27.VDDIO_MEM_S3  pwr
T28.VSS  G$9:T28.VSS  out
T29.VDDIO_MEM_S3  G$8:T29.VDDIO_MEM_S3  pwr
T30.VSS  G$9:T30.VSS  out
T31.MA_ADD[3]  G$1:T31.MA_ADD[3]
T32.MA_ADD[1]  G$1:T32.MA_ADD[1]
T33.VDDIO_MEM_S3  G$8:T33.VDDIO_MEM_S3  pwr
T34.MA_CLK_H[0]  G$1:T34.MA_CLK_H[0]
T35.MA_ADD[2]  G$1:T35.MA_ADD[2]
T36.VDDIO_MEM_S3  G$8:T36.VDDIO_MEM_S3  pwr
T37.MB_ADD[4]  G$2:T37.MB_ADD[4]
T38.MB_ADD[3]  G$2:T38.MB_ADD[3]
T39.VDDIO_MEM_S3  G$8:T39.VDDIO_MEM_S3  pwr
U1.P_GFX_TXN[12]  G$5:U1.P_GFX_TXN[12]
U2.VDDCR_CPU  G$6:U2.VDDCR_CPU  pwr
U3.P_GFX_TXP[13]  G$5:U3.P_GFX_TXP[13]
U4.VSS  G$9:U4.VSS  out
U5.VSS  G$9:U5.VSS  out
U6.P_GFX_RXN[14]  G$5:U6.P_GFX_RXN[14]
U7.P_GFX_RXP[14]  G$5:U7.P_GFX_RXP[14]
U8.VSS  G$9:U8.VSS  out
U9.VSS  G$9:U9.VSS  out
U10.VDDCR_CPU  G$6:U10.VDDCR_CPU  pwr
U11.VSS  G$9:U11.VSS  out
U12.VDDCR_SOC  G$6:U12.VDDCR_SOC  pwr
U13.VSS  G$9:U13.VSS  out
U27.VSS  G$9:U27.VSS  out
U28.VDDIO_MEM_S3  G$8:U28.VDDIO_MEM_S3  pwr
U29.VSS  G$9:U29.VSS  out
U30.VDDIO_MEM_S3  G$8:U30.VDDIO_MEM_S3  pwr
U31.VSS  G$9:U31.VSS  out
U32.VDDIO_MEM_S3  G$8:U32.VDDIO_MEM_S3  pwr
U33.MA_CLK_H[1]  G$1:U33.MA_CLK_H[1]
U34.MA_CLK_L[0]  G$1:U34.MA_CLK_L[0]
U35.VDDIO_MEM_S3  G$8:U35.VDDIO_MEM_S3  pwr
U36.MB_ADD[1]  G$2:U36.MB_ADD[1]
U37.MB_ADD[2]  G$2:U37.MB_ADD[2]
U38.VDDIO_MEM_S3  G$8:U38.VDDIO_MEM_S3  pwr
U39.MB_CLK_H[0]  G$2:U39.MB_CLK_H[0]
V1.VSS  G$9:V1.VSS  out
V2.P_GFX_TXP[14]  G$5:V2.P_GFX_TXP[14]
V3.P_GFX_TXN[13]  G$5:V3.P_GFX_TXN[13]
V4.VSS  G$9:V4.VSS  out
V5.P_GFX_RXN[15]  G$5:V5.P_GFX_RXN[15]
V6.P_GFX_RXP[15]  G$5:V6.P_GFX_RXP[15]
V7.VSS  G$9:V7.VSS  out
V8.P0A_ZVSS  G$5:V8.P0A_ZVSS  out
V9.VDDCR_CPU  G$6:V9.VDDCR_CPU  pwr
V10.VSS  G$9:V10.VSS  out
V11.VDDCR_CPU  G$6:V11.VDDCR_CPU  pwr
V12.VSS  G$9:V12.VSS  out
V13.VDDCR_SOC  G$6:V13.VDDCR_SOC  pwr
V27.VDDIO_MEM_S3  G$8:V27.VDDIO_MEM_S3  pwr
V28.VSS  G$9:V28.VSS  out
V29.VDDIO_MEM_S3  G$8:V29.VDDIO_MEM_S3  pwr
V30.VSS  G$9:V30.VSS  out
V31.VDDIO_MEM_S3  G$8:V31.VDDIO_MEM_S3  pwr
V32.MA_CLK_H[3]  G$1:V32.MA_CLK_H[3]
V33.MA_CLK_L[1]  G$1:V33.MA_CLK_L[1]
V34.VDDIO_MEM_S3  G$8:V34.VDDIO_MEM_S3  pwr
V35.MA_CLK_H[2]  G$1:V35.MA_CLK_H[2]
V36.MA_CLK_L[2]  G$1:V36.MA_CLK_L[2]
V37.VDDIO_MEM_S3  G$8:V37.VDDIO_MEM_S3  pwr
V38.MB_CLK_H[1]  G$2:V38.MB_CLK_H[1]
V39.MB_CLK_L[0]  G$2:V39.MB_CLK_L[0]
W1.P_GFX_TXP[15]  G$5:W1.P_GFX_TXP[15]
W2.P_GFX_TXN[14]  G$5:W2.P_GFX_TXN[14]
W3.VDDCR_CPU  G$6:W3.VDDCR_CPU  pwr
W4.P_HUB_RXP[3]  G$5:W4.P_HUB_RXP[3]
W5.P_HUB_RXN[3]  G$5:W5.P_HUB_RXN[3]
W6.VDDCR_CPU  G$6:W6.VDDCR_CPU  pwr
W7.P_ZVSS  G$5:W7.P_ZVSS  out
W8.P_ZVDDP  G$5:W8.P_ZVDDP  pwr
W9.VSS  G$9:W9.VSS  out
W10.VDDCR_CPU  G$6:W10.VDDCR_CPU  pwr
W11.VSS  G$9:W11.VSS  out
W12.VDDCR_CPU  G$6:W12.VDDCR_CPU  pwr
W13.VSS  G$9:W13.VSS  out
W27.VSS  G$9:W27.VSS  out
W28.VDDIO_MEM_S3  G$8:W28.VDDIO_MEM_S3  pwr
W29.VSS  G$9:W29.VSS  out
W30.TEST40  G$3:W30.TEST40
W31.VSS  G$9:W31.VSS  out
W32.MA_CLK_L[3]  G$1:W32.MA_CLK_L[3]
W33.VDDIO_MEM_S3  G$8:W33.VDDIO_MEM_S3  pwr
W34.VDDIO_MEM_S3  G$8:W34.VDDIO_MEM_S3  pwr
W35.MA_EVENT_L  G$1:W35.MA_EVENT_L
W36.VDDIO_MEM_S3  G$8:W36.VDDIO_MEM_S3  pwr
W37.MB_CLK_H[2]  G$2:W37.MB_CLK_H[2]
W38.MB_CLK_L[1]  G$2:W38.MB_CLK_L[1]
W39.VDDIO_MEM_S3  G$8:W39.VDDIO_MEM_S3  pwr
Y1.P_GFX_TXN[15]  G$5:Y1.P_GFX_TXN[15]
Y2.VDDCR_CPU  G$6:Y2.VDDCR_CPU  pwr
Y3.USB_SS_0RXP  G$4:Y3.USB_SS_0RXP
Y4.USB_SS_0RXN  G$4:Y4.USB_SS_0RXN
Y5.VSS  G$9:Y5.VSS  out
Y6.P_HUB_RXP[2]  G$5:Y6.P_HUB_RXP[2]
Y7.P_HUB_RXN[2]  G$5:Y7.P_HUB_RXN[2]
Y8.VSS  G$9:Y8.VSS  out
Y9.VDDCR_CPU  G$6:Y9.VDDCR_CPU  pwr
Y10.VSS  G$9:Y10.VSS  out
Y11.VDDCR_CPU  G$6:Y11.VDDCR_CPU  pwr
Y12.VSS  G$9:Y12.VSS  out
Y13.VDDCR_CPU  G$6:Y13.VDDCR_CPU  pwr
Y27.VDDIO_MEM_S3  G$8:Y27.VDDIO_MEM_S3  pwr
Y28.VSS  G$9:Y28.VSS  out
Y29.VDDIO_MEM_S3  G$8:Y29.VDDIO_MEM_S3  pwr
Y30.VSS  G$9:Y30.VSS  out
Y31.VDDIO_MEM_S3  G$8:Y31.VDDIO_MEM_S3  pwr
Y32.VDDIO_MEM_S3  G$8:Y32.VDDIO_MEM_S3  pwr
Y33.MA_PARTOUT  G$1:Y33.MA_PARTOUT  out
Y34.MA__ZVDDIO_MEM_S3  G$1:Y34.MA__ZVDDIO_MEM_S3  pwr
Y35.VDDIO_MEM_S3  G$8:Y35.VDDIO_MEM_S3  pwr
Y36.MB__ZVDDIO_MEM_S3  G$2:Y36.MB__ZVDDIO_MEM_S3  pwr
Y37.MB_CLK_L[2]  G$2:Y37.MB_CLK_L[2]
Y38.VDDIO_MEM_S3  G$8:Y38.VDDIO_MEM_S3  pwr
Y39.MB_CLK_H[3]  G$2:Y39.MB_CLK_H[3]

## Footprint AM4_SOCKET (pad centres in mm)
Here is le pièce de résistance, AMD's 1331 pin AM4 Socket in all its glory. I named every pin by hand :P Shaped and Based on the Foxconn PZ1331A-51ZZ0-1H AM4 Socket by the one and only, YeaTheMen
smd 0.485 x 0.485: A3.VSS -17,19; AG1.VSS -19,-7; AH1.X48M_X2 -19,-8; AJ1.X48M_X1 -19,-9; AL1.USB_OC0_L/AGPIO16 -19,-11; AM1.USB_OC1_L/TDI/AGPIO17 -19,-12; AN1.VSS -19,-13; AP1.USB_OC3_L/TDO/AGPIO24 -19,-14; AR1.USB_OC2_L/TCK/AGPIO18 -19,-15; AT1.VSS -19,-16; AU1.AZ_RST_L -19,-17; AV2.VSS -18,-18; AW3.AZ_BITCLK -17,-19; B3.DP0_TXN[1] -17,18; C1.VSS -19,17; D1.P_GFX_TXP[0] -19,16; E1.P_GFX_TXN[0] -19,15; F1.VSS -19,14; G1.P_GFX_TXP[3] -19,13; H1.P_GFX_TXN[3] -19,12; J1.VSS -19,11; L1.P_GFX_TXN[6] -19,9; M1.VSS -19,8; N1.P_GFX_TXP[9] -19,7
smd 0.485 x 0.458: A4.DP0_TXN[2] -16,19; A5.RSVD -15,19; A6.VSS -14,19; A7.DP2_TXP[1] -13,19; A8.DP2_TXN[1] -12,19; A9.VSS -11,19; A10.DP2_AUXP -10,19; A11.DP2_AUXN -9,19; A12.VSS -8,19; A13.TEST11 -7,19; A14.TDI -6,19; A15.VSS -5,19; A16.TEST41 -4,19; A17.SVT -3,19; A18.VSS -2,19; A19.THERMTRIP_L -1,19; A20.MB_DATA[4] 0,19; A21.VSS 1,19; A22.MB_DQS_L[0] 2,19; A23.MB_DATA[6] 3,19; A24.VSS 4,19; A25.MB_DATA[12] 5,19; A26.MB_DATA[8] 6,19; A27.VSS 7,19; A28.MB_DATA[14] 8,19; A29.MB_DATA[10] 9,19; A30.VSS 10,19; A31.MB_DATA[16] 11,19; A32.MB_DM[2] 12,19; A33.VSS 13,19; A34.MB_DATA[23] 14,19; A35.MB_DATA[28] 15,19; A36.VSS 16,19; A37.MB_DQS_L[3] 17,19; AA1.VSS -19,-1; AA2.USB_SS_1RXP -18,-1; AA3.USB_SS_1RXN -17,-1; AA4.VSS -16,-1; AA5.P_HUB_TXP[1] -15,-1; AA6.VSS -14,-1; AA7.VDDCR_CPU -13,-1; AA8.P_HUB_RXN[1] -12,-1; AA9.VSS -11,-1; AA10.VDDCR_CPU -10,-1; AA11.VSS -9,-1; AA12.VDDCR_CPU -8,-1; AA13.VSS -7,-1; AA27.VSS 7,-1; AA28.VDDIO_MEM_S3 8,-1; AA29.VSS 9,-1; AA30.TEST31 10,-1; AA31.VSS 11,-1; AA32.MA_ADD[0] 12,-1; AA33.MA_BANK[1] 13,-1; AA34.VDDIO_MEM_S3 14,-1; AA35.MA_BANK[0] 15,-1; AA36.MA_ADD[10] 16,-1; AA37.VDDIO_MEM_S3 17,-1; AA38.MB_EVENT_L 18,-1; AA39.MB_CLK_L[3] 19,-1; AB1.USB_SS_1TXP -19,-2; AB2.RSVD -18,-2; AB3.VDDCR_CPU -17,-2; AB4.TEST10 -16,-2; AB5.P_HUB_TXN[1] -15,-2; AB6.VDDCR_CPU -14,-2; AB7.VSS -13,-2; AB8.P_HUB_RXP[1] -12,-2; AB9.VDDCR_CPU -11,-2; AB10.VSS -10,-2; AB11.VDDCR_CPU -9,-2; AB12.VSS -8,-2; AB13.VDDCR_CPU -7,-2; AB27.VDDIO_MEM_S3 7,-2; AB28.VSS 8,-2; AB29.VDDIO_MEM_S3 9,-2; AB30.VSS 10,-2; AB31.VDDIO_MEM_S3 11,-2; AB32.VDDIO_MEM_S3 12,-2; AB33.VDDIO_MEM_S3 13,-2; AB34.MA_RAS_L_ADD[16] 14,-2; AB35.MA_WE_L_ADD[14] 15,-2; AB36.VDDIO_MEM_S3 16,-2; AB37.RSVD 17,-2; AB38.MB_PARTOUT 18,-2; AB39.VDDIO_MEM_S3 19,-2; AC1.USB_SS_1TXN -19,-3; AC2.VDDCR_CPU -18,-3; AC3.USB_SS_2TXP -17,-3; AC4.USB_SS_2TXN -16,-3; AC5.VSS -15,-3; AC6.P_HUB_TXP[2] -14,-3; AC7.P_HUB_TXN[2] -13,-3; AC8.VSS -12,-3; AC9.VSS -11,-3; AC10.VDDCR_CPU -10,-3; AC11.VSS -9,-3; AC12.VDDCR_CPU -8,-3; AC13.VSS -7,-3; AC27.VSS 7,-3; AC28.VDDIO_MEM_S3 8,-3; AC29.VSS 9,-3; AC30.VDDIO_MEM_S3 10,-3; AC31.VSS 11,-3; AC32.VDDIO_MEM_S3 12,-3; AC33.MA0_CS_L[0] 13,-3; AC34.MA1_CS_L[0] 14,-3; AC35.VDDIO_MEM_S3 15,-3; AC36.MB_ADD[0] 16,-3; AC37.MB_BANK[1] 17,-3; AC38.VDDIO_MEM_S3 18,-3; AC39.MB_ADD[10] 19,-3; AD1.VSS -19,-4; AD2.USB_SS_3RXP -18,-4; AD3.RSVD -17,-4; AD4.VSS -16,-4; AD5.P_HUB_TXP[3] -15,-4; AD6.P_HUB_TXN[3] -14,-4; AD7.VDDCR_CPU -13,-4; AD8.P_HUB_RXN[0] -12,-4; AD9.VDDCR_CPU -11,-4; AD10.VSS -10,-4; AD11.VDDCR_CPU -9,-4; AD12.VSS -8,-4; AD13.VDDCR_CPU -7,-4; AD27.VDDIO_MEM_S3 7,-4; AD28.VSS 8,-4; AD29.VDDIO_MEM_S3 9,-4; AD30.VSS 10,-4; AD31.VDDIO_MEM_S3 11,-4; AD32.MA_CAS_L_ADD[15] 12,-4; AD33.MA1_ODT[0] 13,-4; AD34.VDDIO_MEM_S3 14,-4; AD35.MA0_ODT[0] 15,-4; AD36.MB_RAS_L_ADD[16] 16,-4; AD37.VDDIO_MEM_S3 17,-4; AD38.MB_BANK[0] 18,-4; AD39.MB_WE_L_ADD[14] 19,-4; AE1.USB_SS_3RXP -19,-5; AE2.USB_SS_2RXN -18,-5; AE3.VDDCR_CPU -17,-5; AE4.P_HUB_TXP[0] -16,-5; AE5.P_HUB_TXN[0] -15,-5; AE6.VDDCR_CPU -14,-5; AE7.VSS -13,-5; AE8.P_HUB_RXP[0] -12,-5; AE9.VSS -11,-5; AE10.VDDCR_CPU -10,-5; AE11.VSS -9,-5; AE12.VDDCR_CPU -8,-5; AE13.VSS -7,-5; AE27.VSS 7,-5; AE28.VDDIO_MEM_S3 8,-5; AE29.VSS 9,-5; AE30.VDDIO_MEM_S3 10,-5; AE31.VSS 11,-5; AE32.MA_ADD[13] 12,-5; AE33.VDDIO_MEM_S3 13,-5; AE34.MA1_CS_L[1] 14,-5; AE35.MA0_CS_L[1] 15,-5; AE36.VDDIO_MEM_S3 16,-5; AE37.MB0_CS_L[0] 17,-5; AE38.MB1_CS_L[0] 18,-5; AE39.VDDIO_MEM_S3 19,-5; AF1.USB_SS_3RXN -19,-6; AF2.VDDCR_CPU -18,-6; AF3.USB_SS_0TXP -17,-6; AF4.USB_SS_0TXN -16,-6; AF5.VSS -15,-6; AF6.GFX_CLKP -14,-6; AF7.GFX_CLKN -13,-6; AF8.VSS -12,-6; AF9.VDDCR_CPU -11,-6; AF10.VSS -10,-6; AF11.VDDCR_CPU -9,-6; AF12.VSS -8,-6; AF13.VDDCR_CPU -7,-6; AF27.VDDIO_MEM_S3 7,-6; AF28.VSS 8,-6; AF29.VDDIO_MEM_S3 9,-6; AF30.VSS 10,-6; AF31.MA0_ODT[1] 11,-6; AF32.VDDIO_MEM_S3 12,-6; AF33.MA_ADD_17 13,-6; AF34.MA1_ODT[1] 14,-6; AF35.VDDIO_MEM_S3 15,-6; AF36.MB_CAS_L_ADD[15] 16,-6; AF37.MB1_ODT[0] 17,-6; AF38.VDDIO_MEM_S3 18,-6; AF39.MB0_ODT[0] 19,-6; AG2.USB_SS_3TXP -18,-7; AG3.USB_SS_3TXN -17,-7; AG4.VSS -16,-7; AG5.GPP_CLK0P -15,-7; AG6.GPP_CLK0N -14,-7; AG7.VDDCR_CPU -13,-7; AG8.VSS -12,-7; AG9.VSS -11,-7; AG10.VDDCR_CPU -10,-7; AG11.VSS -9,-7; AG12.VDDCR_CPU -8,-7; AG13.VSS -7,-7; AG14.VDDCR_CPU -6,-7; AG15.VSS -5,-7; AG16.VDDCR_CPU -4,-7; AG17.VSS -3,-7; AG18.VDDCR_CPU -2,-7; AG19.VSS -1,-7; AG20.VDDCR_CPU 0,-7; AG21.VSS 1,-7; AG22.VDDCR_CPU 2,-7; AG23.VSS 3,-7; AG24.VDDCR_CPU 4,-7; AG25.VSS 5,-7; AG26.VDDCR_CPU 6,-7; AG27.VSS 7,-7; AG28.VSS 8,-7; AG29.VSS 9,-7; AG30.VSS 10,-7; AG31.VSS 11,-7; AG32.VSS 12,-7; AG33.VDDIO_MEM_S3 13,-7; AG34.VDDIO_MEM_S3 14,-7; AG35.VDDIO_MEM_S3 15,-7; AG36.MB1_CS_L[1] 16,-7; AG37.VDDIO_MEM_S3 17,-7; AG38.MB_ADD[13] 18,-7; AG39.MB0_CS_L[1] 19,-7; AH2.RSVD -18,-8; AH3.VDDCR_CPU -17,-8; AH4.GPP_CLK1P -16,-8; AH5.GPP_CLK1N -15,-8; AH6.VDDCR_CPU -14,-8; AH7.GPP_CLK2P -13,-8; AH8.GPP_CLK2N -12,-8; AH9.VDDCR_CPU -11,-8; AH10.VSS -10,-8; AH11.VDDCR_CPU -9,-8; AH12.VSS -8,-8; AH13.VDDCR_CPU -7,-8; AH14.VSS -6,-8; AH15.VDDCR_CPU -5,-8; AH16.VSS -4,-8; AH17.VDDCR_CPU -3,-8; AH18.VSS -2,-8; AH19.VDDCR_CPU -1,-8; AH20.VSS 0,-8; AH21.VDDCR_CPU 1,-8; AH22.VSS 2,-8; AH23.VDDCR_CPU 3,-8; AH24.VSS 4,-8; AH25.VDDCR_CPU 5,-8; AH26.VSS 6,-8; AH27.VDDCR_CPU 7,-8; AH28.VSS 8,-8; AH29.VSS 9,-8; AH30.VSS 10,-8; AH31.MA_DATA[36] 11,-8; AH32.MA_DATA[37] 12,-8; AH33.VSS 13,-8; AH34.MA_DATA[32] 14,-8; AH35.RSVD 15,-8; AH36.MB0_ODT[1] 16,-8; AH37.MB_ADD_17 17,-8; AH38.MB1_ODT[1] 18,-8; AH39.VDDIO_MEM_S3 19,-8; AJ2.VDDCR_CPU -18,-9; AJ3.USB0_ZVSS -17,-9; AJ4.USB_SS_ZVSS -16,-9; AJ5.VSS -15,-9; AJ6.GPP_CLK3P -14,-9; AJ7.GPP_CLK3N -13,-9; AJ8.VSS -12,-9; AJ9.VSS -11,-9; AJ10.VDDCR_CPU -10,-9; AJ11.VSS -9,-9; AJ12.VDDCR_CPU -8,-9; AJ13.VSS -7,-9; AJ14.VDDCR_CPU -6,-9; AJ15.VDD_18_S5 -5,-9; AJ16.VDDP_S5 -4,-9; AJ17.VDDP_S5 -3,-9; AJ18.VDDCR_SOC_S5 -2,-9; AJ19.VDD_33_S5 -1,-9; AJ20.VDD_18 0,-9; AJ21.VDD_33 1,-9; AJ22.VDDCR_CPU 2,-9; AJ23.VSS 3,-9; AJ24.VDDCR_CPU 4,-9; AJ25.VSS 5,-9; AJ26.VSS 6,-9; AJ27.VSS 7,-9; AJ28.VSS 8,-9; AJ29.VSS 9,-9; AJ30.MA_DATA[33] 10,-9; AJ31.MA_DM[4] 11,-9; AJ32.VSS 12,-9; AJ33.MA_DQS_H[4] 13,-9; AJ34.MA_DQS_L[4] 14,-9; AJ35.VSS 15,-9; AJ36.VSS 16,-9; AJ37.MA_ZVSS 17,-9; AJ38.VSS 18,-9; AJ39.MB_ZVSS 19,-9; AK1.VSS -19,-10; AK2.SDA1/I2C3_SDA/AGPIO20 -18,-10; AK3.SCL1/I2C3_SCL/AGPIO19 -17,-10; AK4.VSS -16,-10; AK5.USB3_ZVSS -15,-10; AK6.USB2_ZVSS -14,-10; AK7.VDDCR_CPU -13,-10; AK8.USB_SS_ZVDDP -12,-10; AK9.VDDCR_CPU -11,-10; AK10.VSS -10,-10; AK11.VDDCR_CPU -9,-10; AK12.VSS -8,-10; AK13.VDDCR_CPU -7,-10; AK14.VSS -6,-10; AK15.VDD_18_S5 -5,-10; AK18.VDDCR_SOC_S5 -2,-10; AK19.VDD_33_S5 -1,-10; AK20.VDD_18 0,-10; AK21.VDD_33 1,-10; AK22.VSS 2,-10; AK25.VSS 5,-10; AK26.MA_DATA[57] 6,-10; AK27.MA_DATA[56] 7,-10; AK28.VSS 8,-10; AK29.MA_DATA[49] 9,-10; AK30.MA_DATA[34] 10,-10; AK31.VSS 11,-10; AK32.MA_DATA[39] 12,-10; AK33.MA_DATA[38] 13,-10; AK34.RSVD 14,-10; AK35.VSS 15,-10; AK36.MB_DATA[37] 16,-10; AK37.VSS 17,-10; AK38.MB_DATA[36] 18,-10; AK39.MB_DATA[32] 19,-10; AL2.LPC_PME_L/AGPIO22 -18,-11; AL3.VDDCR_CPU -17,-11; AL4.TEST46[13] -16,-11; AL5.WAKE_L/AGPIO2 -15,-11; AL6.VDDCR_CPU -14,-11; AL7.PCIE_RST_L/EGPIO26 -13,-11; AL8.AM4R1 -12,-11; AL9.VSS -11,-11; AL10.VDDCR_CPU -10,-11; AL11.VSS -9,-11; AL12.VDDCR_CPU -8,-11; AL13.P_GPP_TXP[2]/SATA_TX0P -7,-11; AL14.VDDCR_CPU -6,-11; AL15.VDDBT_RTC_G -5,-11; AL16.RSVD -4,-11; AL17.RSVD -3,-11; AL18.RSVD -2,-11; AL19.RSVD -1,-11; AL20.RSVD 0,-11; AL21.RSVD 1,-11; AL22.VDDP_SENSE 2,-11; AL23.CLK_REQ3_L/SATA_IS1_L/SATA_ZP1_L/EGPIO131 3,-11; AL24.VSS 4,-11; AL25.MA_DATA[62] 5,-11; AL26.MA_DM[7] 6,-11; AL27.VSS 7,-11; AL28.MA_DATA[51] 8,-11; AL29.MA_DM[6] 9,-11; AL30.VSS 10,-11; AL31.MA_DATA[45] 11,-11; AL32.MA_DATA[44] 12,-11; AL33.VSS 13,-11; AL34.MA_DATA[35] 14,-11; AL35.VSS 15,-11; AL36.VSS 16,-11; AL37.MB_DATA[33] 17,-11; AL38.MB_DM[4] 18,-11; AL39.VSS 19,-11; AM2.VDDCR_CPU -18,-12; AM3.PWR_GOOD -17,-12; AM4.SYS_RESET_L/AGPIO1 -16,-12; AM5.VSS -15,-12; AM6.TEST0 -14,-12; AM7.TEST1/TMS -13,-12; AM8.VDDCR_CPU -12,-12; AM9.P_GPP_RXP[1] -11,-12; AM10.P_GPP_RXN[1] -10,-12; AM11.VSS -9,-12; AM12.RSVD -8,-12; AM13.P_GPP_TXN[2]/SATA_TX0N -7,-12; AM14.VSS -6,-12; AM15.VDDIO_AUDIO -5,-12; AM16.RSVD -4,-12; AM17.RSVD -3,-12; AM18.VDDP -2,-12; AM19.VDDP -1,-12; AM20.VDDP 0,-12; AM21.RSVD 1,-12; AM22.SATA_ACT_L/AGPIO130 2,-12; AM23.VSS_SENSE_B 3,-12; AM24.CORETYPE[0] 4,-12; AM25.MA_DATA[63] 5,-12; AM26.VSS 6,-12; AM27.MA_DATA[61] 7,-12; AM28.MA_DATA[50] 8,-12; AM29.VSS 9,-12; AM30.MA_DATA[52] 10,-12; AM31.MA_DM[5] 11,-12; AM32.VSS 12,-12; AM33.MA_DATA[41] 13,-12; AM34.MA_DATA[40] 14,-12; AM35.VSS 15,-12; AM36.MB_DQS_L[4] 16,-12; AM37.MB_DQS_H[4] 17,-12; AM38.VSS 18,-12; AM39.MB_DATA[38] 19,-12; AN2.AGPIO9/SGPIO0_DATAOUT -18,-13; AN3.AGPIO23/SGPIO0_LOAD -17,-13; AN4.VSS -16,-13; AN5.PWR_BTN_L/AGPIO0 -15,-13; AN6.USB1_ZVSS -14,-13; AN7.VDDCR_CPU -13,-13; AN8.AGPIO6 -12,-13; AN9.CORETYPE[1] -11,-13; AN10.VDDCR_CPU -10,-13; AN11.P_GPP_RXN[3]/SATA_RX1N -9,-13; AN12.RSVD -8,-13; AN13.VDDCR_CPU -7,-13; AN14.P_GPP_TXP[3]/SATA_TX1P -6,-13; AN15.RSVD -5,-13; AN16.RSVD -4,-13; AN17.RSVD -3,-13; AN18.VDDP -2,-13; AN19.VDDP -1,-13; AN20.VDDP 0,-13; AN21.RSVD 1,-13; AN22.VSS 2,-13; AN23.FANIN0/AGPIO84 3,-13; AN24.ESPI_RESET_L/KBRST_L 4,-13; AN25.VSS 5,-13; AN26.MA_DQS_L[7] 6,-13; AN27.MA_DATA[60] 7,-13; AN28.VSS 8,-13; AN29.MA_DQS_L[6] 9,-13; AN30.MA_DATA[53] 10,-13; AN31.VSS 11,-13; AN32.MA_DQS_H[5] 12,-13; AN33.MA_DQS_L[5] 13,-13; AN34.VSS 14,-13; AN35.VSS 15,-13; AN36.MB_DATA[34] 16,-13; AN37.VSS 17,-13; AN38.MB_DATA[39] 18,-13; AN39.MB_DATA[35] 19,-13; AP2.SLP_S5_L -18,-14; AP3.VDDCR_CPU -17,-14; AP4.S5_MUX_CTRL/EGPIO42 -16,-14; AP5.RSMRST_L -15,-14; AP6.VSS -14,-14; AP7.AGPIO8 -13,-14; AP8.RTCCLK -12,-14; AP9.VDDCR_CPU -11,-14; AP10.P_GPP_RXN[2]/SATA_RX0N -10,-14; AP11.P_GPP_RXP[3]/SATA_RX1P -9,-14; AP12.VDDCR_CPU -8,-14; AP13.P_GPP_TXP[1] -7,-14; AP14.P_GPP_TXN[3]/SATA_TX1N -6,-14; AP15.RSVD -5,-14; AP16.RSVD -4,-14; AP17.RSVD -3,-14; AP18.VDDP -2,-14; AP19.VDDP -1,-14; AP20.VDDP 0,-14; AP21.RSVD 1,-14; AP22.AGPIO5/DEVSLP0 2,-14; AP23.FANOUT0/AGPIO85 3,-14; AP24.VSS 4,-14; AP25.MA_DATA[58] 5,-14; AP26.MA_DQS_H[7] 6,-14; AP27.VSS 7,-14; AP28.MA_DATA[54] 8,-14; AP29.MA_DQS_H[6] 9,-14; AP30.VSS 10,-14; AP31.MA_DATA[42] 11,-14; AP32.MA_DATA[47] 12,-14; AP33.VSS 13,-14; AP34.MA_DATA[46] 14,-14; AP35.VSS 15,-14; AP36.VSS 16,-14; AP37.MB_DATA[44] 17,-14; AP38.MB_DATA[45] 18,-14; AP39.VSS 19,-14; AR2.VDDCR_CPU -18,-15; AR3.S0A3_GPIO/AGPIO10/SGPIO0_CLK -17,-15; AR4.AGPIO40/SGPIO0_DATAIN -16,-15; AR5.VSS -15,-15; AR6.AGPIO4 -14,-15; AR7.48M_OSC -13,-15; AR8.VSS -12,-15; AR9.P_GPP_RXP[0] -11,-15; AR10.P_GPP_RXP[2]/SATA_RX0P -10,-15; AR11.VSS -9,-15; AR12.P_GPP_TXN[0] -8,-15; AR13.P_GPP_TXN[1] -7,-15; AR14.VSS -6,-15; AR15.RSVD -5,-15; AR16.RSVD -4,-15; AR17.VSS -3,-15; AR18.RSVD -2,-15; AR19.RSVD -1,-15; AR20.RSVD 0,-15; AR21.RSVD 1,-15; AR22.CLK_REQG_L/OSCIN/EGPIO132 2,-15; AR23.VSS 3,-15; AR24.RSVD 4,-15; AR25.MA_DATA[59] 5,-15; AR26.VSS 6,-15; AR27.VSS 7,-15; AR28.MA_DATA[55] 8,-15; AR29.VSS 9,-15; AR30.VSS 10,-15; AR31.MA_DATA[48] 11,-15; AR32.VSS 12,-15; AR33.MA_DATA[43] 13,-15; AR34.VSS 14,-15; AR35.VSS 15,-15; AR36.MB_DATA[40] 16,-15; AR37.MB_DATA[41] 17,-15; AR38.VSS 18,-15; AR39.MB_DM[5] 19,-15; AT2.SLP_S3_L -18,-16; AT3.TEST2 -17,-16; AT4.VDDCR_CPU -16,-16; AT5.BLINK/AGPIO11 -15,-16; AT6.AGPIO3 -14,-16; AT7.VSS -13,-16; AT8.P0B_ZVSS -12,-16; AT9.P_GPP_RXN[0] -11,-16; AT10.VSS -10,-16; AT11.USB_ZVSS -9,-16; AT12.P_GPP_TXP[0] -8,-16; AT13.VSS -7,-16; AT14.EGPIO100 -6,-16; AT15.ESPI_ALERT_L/LDRQ0_L/EGPIO108 -5,-16; AT16.VSS -4,-16; AT17.SPI_CS1_L/EGPIO118 -3,-16; AT18.EGPIO70 -2,-16; AT19.RSVD -1,-16; AT20.LAD3/EGPIO107 0,-16; AT21.LAD2/EGPIO106 1,-16; AT22.VSS 2,-16; AT23.CLK_REQ0_L/SATA_IS0_L/SATA_ZP0_L/AGPIO92 3,-16; AT24.CLK_REQ2_L/AGPIO116 4,-16; AT25.RSVD 5,-16; AT26.VSS 6,-16; AT27.VSS 7,-16; AT28.VSS 8,-16; AT29.VSS 9,-16; AT30.RSVD 10,-16; AT31.VSS 11,-16; AT32.VSS 12,-16; AT33.VSS 13,-16; AT34.VSS 14,-16; AT35.MB_DM[6] 15,-16; AT36.MB_DATA[46] 16,-16; AT37.VSS 17,-16; AT38.MB_DQS_H[5] 18,-16; AT39.MB_DQS_L[5] 19,-16; AU2.AZ_SYNC -18,-17; AU3.VDDCR_CPU -17,-17; AU4.AZ_SDOUT -16,-17; AU5.AZ_SDIN1 -15,-17; AU6.VDDCR_CPU -14,-17; AU7.USB_HSD0P -13,-17; AU8.USB_HSD0N -12,-17; AU9.VDDCR_CPU -11,-17; AU10.USB_HSD2P -10,-17; AU11.USB_HSD2N -9,-17; AU12.VDDCR_CPU -8,-17; AU13.EGPIO98 -7,-17; AU14.SPI_DI/ESPI_DAT1/EGPIO120 -6,-17; AU15.VDDCR_CPU -5,-17; AU16.SPI_DO/ESPI_DAT0/EGPIO121 -4,-17; AU17.SPI_TPM_CS_L/AGPIO76 -3,-17; AU18.VSS -2,-17; AU19.LPCCLK1/EGPIO75 -1,-17; AU20.LPCCLK0/EGPIO74 0,-17; AU21.VSS 1,-17; AU22.LPC_RST_L 2,-17; AU23.GENINT2_L/AGPIO90 3,-17; AU24.VSS 4,-17; AU25.SCL0/I2C2_SCL/EGPIO113 5,-17; AU26.VSS 6,-17; AU27.VSS 7,-17; AU28.MB_DQS_H[7] 8,-17; AU29.MB_DQS_L[7] 9,-17; AU30.VSS 10,-17; AU31.MB_DATA[61] 11,-17; AU32.MB_DATA[51] 12,-17; AU33.VSS 13,-17; AU34.MB_DQS_H[6] 14,-17; AU35.MB_DATA[49] 15,-17; AU36.VSS 16,-17; AU37.MB_DATA[42] 17,-17; AU38.MB_DATA[47] 18,-17; AU39.VSS 19,-17; AV3.AZ_SDIN0 -17,-18; AV4.AZ_SDIN2 -16,-18; AV5.VDDCR_CPU -15,-18; AV6.SATA_ZVSS -14,-18; AV7.SATA_ZVDDP -13,-18; AV8.VDDCR_CPU -12,-18; AV9.USB_HSD3P -11,-18; AV10.USB_HSD3N -10,-18; AV11.VDDCR_CPU -9,-18; AV12.EGPIO96 -8,-18; AV13.EGPIO99 -7,-18; AV14.VDDCR_CPU -6,-18; AV15.SPI_HOLD_L/ESPI_DAT3/EGPIO133 -5,-18; AV16.SPI_WP_L/ESPI_DAT2/EGPIO122 -4,-18; AV17.VSS -3,-18; AV18.LPC_PD_L/AGPIO21 -2,-18; AV19.LPC_CLKRUN_L/AGPIO88 -1,-18; AV20.VSS 0,-18; AV21.LAD1/EGPIO105 1,-18; AV22.GENINT1_L/AGPIO89 2,-18; AV23.VSS 3,-18; AV24.CLK_REQ1_L/AGPIO115 4,-18; AV25.SDA0/I2C2_SDA/EGPIO114 5,-18; AV26.VSS 6,-18; AV27.MB_DATA[63] 7,-18; AV28.MB_DATA[62] 8,-18; AV29.VSS 9,-18; AV30.MB_DATA[57] 10,-18; AV31.MB_DATA[60] 11,-18; AV32.VSS 12,-18; AV33.MB_DATA[55] 13,-18; AV34.MB_DQS_L[6] 14,-18; AV35.VSS 15,-18; AV36.MB_DATA[52] 16,-18; AV37.MB_DATA[43] 17,-18; AV38.VSS 18,-18; AW4.VSS -16,-19; AW5.X32K_X1 -15,-19; AW6.X32K_X2 -14,-19; AW7.VSS -13,-19; AW8.USB_HSD1P -12,-19; AW9.USB_HSD1N -11,-19; AW10.VSS -10,-19; AW11.EGPIO95 -9,-19; AW12.EGPIO97 -8,-19; AW13.VSS -7,-19; AW14.SPI_CLK/ESPI_CLK/EGPIO117 -6,-19; AW15.SPI_CS2_L/ESPI_CS_L/EGPIO119 -5,-19; AW16.VSS -4,-19; AW17.AGPIO86 -3,-19; AW18.LFRAME_L/EGPIO109 -2,-19; AW19.VSS -1,-19; AW20.LAD0/EGPIO104 0,-19; AW21.SERIRQ/AGPIO87 1,-19; AW22.VSS 2,-19; AW23.SPKR/AGPIO91 3,-19; AW24.RSVD 4,-19; AW25.VSS 5,-19; AW26.MB_DATA[59] 6,-19; AW27.MB_DATA[58] 7,-19; AW28.VSS 8,-19; AW29.MB_DM[7] 9,-19; AW30.MB_DATA[56] 10,-19; AW31.VSS 11,-19; AW32.MB_DATA[50] 12,-19; AW33.MB_DATA[54] 13,-19; AW34.VSS 14,-19; AW35.MB_DATA[48] 15,-19; AW36.MB_DATA[53] 16,-19; AW37.VSS 17,-19; B4.DP0_TXP[2] -16,18; B5.VDDCR_SOC -15,18; B6.DP2_TXP[0] -14,18; B7.DP2_TXN[0] -13,18; B8.VDDCR_SOC -12,18; B9.DP2_TXP[3] -11,18; B10.DP2_TXN[3] -10,18; B11.VDDCR_SOC -9,18; B12.TEST15 -8,18; B13.TRST_L -7,18; B14.VDDCR_SOC -6,18; B15.TMS -5,18; B16.RESET_L -4,18; B17.VDDCR_SOC -3,18; B18.SIC -2,18; B19.VSS -1,18; B20.VDDCR_SOC 0,18; B21.MB_DATA[1] 1,18; B22.MB_DQS_H[0] 2,18; B23.VSS 3,18; B24.MB_DATA[2] 4,18; B25.MB_DATA[13] 5,18; B26.VSS 6,18; B27.MB_DQS_L[1] 7,18; B28.MB_DATA[15] 8,18; B29.VSS 9,18; B30.MB_DATA[20] 10,18; B31.MB_DATA[17] 11,18; B32.VSS 12,18; B33.MB_DATA[22] 13,18; B34.MB_DATA[18] 14,18; B35.VSS 15,18; B36.MB_DATA[24] 16,18; B37.MB_DQS_H[3] 17,18; B38.MB_DATA[30] 18,18; C2.DP0_TXN[0] -18,17; C3.DP0_TXP[1] -17,17; C4.VDDCR_SOC -16,17; C5.DP0_TXP[3] -15,17; C6.DP0_TXN[3] -14,17; C7.VDDCR_SOC -13,17; C8.DP2_TXP[2] -12,17; C9.DP2_TXN[2] -11,17; C10.VDDCR_SOC -10,17; C11.TEST16 -9,17; C12.TEST14 -8,17; C13.VDDCR_SOC -7,17; C14.TDO -6,17; C15.TCK -5,17; C16.VDDCR_SOC -4,17; C17.SVD -3,17; C18.SID -2,17; C19.VDDCR_SOC -1,17; C20.MB_DATA[5] 0,17; C21.MB_DM[0] 1,17; C22.VSS 2,17; C23.MB_DATA[7] 3,17; C24.MB_DATA[3] 4,17; C25.VSS 5,17; C26.MB_DATA[9] 6,17; C27.MB_DQS_H[1] 7,17; C28.VSS 8,17; C29.MB_DATA[11] 9,17; C30.MB_DATA[21] 10,17; C31.VSS 11,17; C32.MB_DQS_L[2] 12,17; C33.MB_DQS_H[2] 13,17; C34.VSS 14,17; C35.MB_DATA[19] 15,17; C36.MB_DATA[29] 16,17; C37.VSS 17,17; C38.MB_DATA[31] 18,17; C39.MB_DATA[26] 19,17; D2.DP0_TXP[0] -18,16; D3.VDDCR_SOC -17,16; D4.DP1_TXP[0] -16,16; D5.DP1_TXN[0] -15,16; D6.VSS -14,16; D7.DP1_TXP[1] -13,16; D8.DP1_TXN[1] -12,16; D9.VSS -11,16; D10.DP1_HPD -10,16; D11.TEST17 -9,16; D12.VSS -8,16; D13.TEST6 -7,16; D14.DBREQ_L -6,16; D15.VSS -5,16; D16.ALERT_L -4,16; D17.SVC -3,16; D18.VSS -2,16; D19.VSS -1,16; D20.MB_DATA[0] 0,16; D21.VSS 1,16; D22.VSS 2,16; D23.VSS 3,16; D24.VSS 4,16; D25.VSS 5,16; D26.MB_DM[1] 6,16; D27.VSS 7,16; D28.RSVD 8,16; D29.VSS 9,16; D30.VSS 10,16; D31.VSS 11,16; D32.VSS 12,16; D33.VSS 13,16; D34.VSS 14,16; D35.VSS 15,16; D36.VSS 16,16; D37.MB_DM[3] 17,16; D38.MB_DATA[27] 18,16; D39.VSS 19,16; E2.VDDCR_SOC -18,15; E3.P_GFX_TXP[1] -17,15; E4.VSS -16,15; E5.VSS -15,15; E6.TEST28_H -14,15; E7.TEST28_L -13,15; E8.VSS -12,15; E9.DP1_TXP[3] -11,15; E10.DP2_HPD -10,15; E11.VSS -9,15; E12.DP_AUX_ZVSS -8,15; E13.DBRDY -7,15; E14.VSS -6,15; E15.VDDCR_SOC_SENSE -5,15; E16.PWROK -4,15; E17.VSS -3,15; E18.MA_DATA[0] -2,15; E19.RSVD -1,15; E20.VSS 0,15; E21.VSS 1,15; E22.RSVD 2,15; E23.VSS 3,15; E24.MA_DATA[10] 4,15; E25.RSVD 5,15; E26.VSS 6,15; E27.VSS 7,15; E28.MA_DATA[22] 8,15; E29.VSS 9,15; E30.MA_DQS_L[3] 10,15; E31.MA_DATA[30] 11,15; E32.VSS 12,15; E33.MA_CHECK[4] 13,15; E34.MA_CHECK[5] 14,15; E35.VSS 15,15; E36.MB_DATA[25] 16,15; E37.MB_CHECK[4] 17,15; E38.VSS 18,15; E39.MB_CHECK[5] 19,15; F2.P_GFX_TXP[2] -18,14; F3.P_GFX_TXN[1] -17,14; F4.VSS -16,14; F5.P_GFX_RXN[0] -15,14; F6.P_GFX_RXP[0] -14,14; F7.VDDCR_SOC -13,14; F8.DP1_TXP[2] -12,14; F9.DP1_TXN[3] -11,14; F10.VDDCR_SOC -10,14; F11.DP1_AUXP -9,14; F12.DP_ZVSS -8,14; F13.VDDCR_SOC -7,14; F14.VDDCR_CPU_SENSE -6,14; F15.VSS_SENSE_A -5,14; F16.VDDCR_SOC -4,14; F17.VSS -3,14; F18.MA_DATA[5] -2,14; F19.VSS -1,14; F20.MA_DATA[7] 0,14; F21.MA_DATA[12] 1,14; F22.VSS 2,14; F23.MA_DQS_H[1] 3,14; F24.MA_DATA[15] 4,14; F25.VSS 5,14; F26.MA_DQS_L[2] 6,14; F27.MA_DQS_H[2] 7,14; F28.VSS 8,14; F29.MA_DATA[24] 9,14; F30.MA_DQS_H[3] 10,14; F31.VSS 11,14; F32.MA_DATA[27] 12,14; F33.MA_CHECK[0] 13,14; F34.VSS 14,14; F35.VSS 15,14; F36.MB_CHECK[1] 16,14; F37.VSS 17,14; F38.MB_CHECK[0] 18,14; F39.MB_DM[8] 19,14; G2.P_GFX_TXN[2] -18,13; G3.VDDCR_SOC -17,13; G4.P_GFX_RXN[1] -16,13; G5.P_GFX_RXP[1] -15,13; G6.VDDCR_SOC -14,13; G7.VSS -13,13; G8.DP1_TXN[2] -12,13; G9.VDDCR_SOC -11,13; G10.DP0_AUXP -10,13; G11.DP1_AUXN -9,13; G12.VDDCR_SOC -8,13; G13.DP_BLON -7,13; G14.VDDIO_MEM_S3_SENSE -6,13; G15.VDDCR_SOC -5,13; G16.TEST18 -4,13; G17.RSVD -3,13; G18.VDDCR_SOC -2,13; G19.MA_DQS_L[0] -1,13; G20.MA_DATA[6] 0,13; G21.VSS 1,13; G22.MA_DATA[9] 2,13; G23.MA_DQS_L[1] 3,13; G24.VSS 4,13; G25.MA_DATA[21] 5,13; G26.MA_DM[2] 6,13; G27.VSS 7,13; G28.MA_DATA[18] 8,13; G29.MA_DATA[29] 9,13; G30.VSS 10,13; G31.MA_DATA[31] 11,13; G32.MA_CHECK[1] 12,13; G33.VSS 13,13; G34.MA_DM[8] 14,13; G35.VSS 15,13; G36.VSS 16,13; G37.MB_DQS_L[8] 17,13; G38.MB_DQS_H[8] 18,13; G39.VSS 19,13; H2.VDDCR_SOC -18,12; H3.P_GFX_TXP[4] -17,12; H4.VSS -16,12; H5.VSS -15,12; H6.P_GFX_RXN[2] -14,12; H7.P_GFX_RXP[2] -13,12; H8.VSS -12,12; H9.DP0_HPD -11,12; H10.DP0_AUXN -10,12; H11.VSS -9,12; H12.DP_VARYBL -8,12; H13.DP_DIGON -7,12; H14.VSS -6,12; H15.PROCHOT_L -5,12; H16.TEST19 -4,12; H17.VSS -3,12; H18.MA_DATA[4] -2,12; H19.MA_DQS_H[0] -1,12; H20.VSS 0,12; H21.MA_DATA[3] 1,12; H22.MA_DATA[8] 2,12; H23.VSS 3,12; H24.MA_DATA[14] 4,12; H25.MA_DATA[20] 5,12; H26.VSS 6,12; H27.MA_DATA[23] 7,12; H28.MA_DATA[19] 8,12; H29.VSS 9,12; H30.MA_DM[3] 10,12; H31.MA_DATA[26] 11,12; H32.VSS 12,12; H33.MA_DQS_L[8] 13,12; H34.MA_DQS_H[8] 14,12; H35.VSS 15,12; H36.MB_CHECK[6] 16,12; H37.MB_CHECK[7] 17,12; H38.VSS 18,12; H39.MB_CHECK[2] 19,12; J2.P-GFX_TXP[5] -18,11; J3.P_GFX_TXN[4] -17,11; J4.VSS -16,11; J5.P_GFX_RXN[3] -15,11; J6.P_GFX_RXP[3] -14,11; J7.VDDCR_SOC -13,11; J8.VSS -12,11; J9.VSS -11,11; J10.VDDCR_SOC -10,11; J11.VSS -9,11; J12.VDDCR_SOC -8,11; J13.VSS -7,11; J14.VDDCR_SOC -6,11; J15.VSS -5,11; J16.VDDCR_SOC -4,11; J17.VSS -3,11; J18.MA_DATA[1] -2,11; J19.VSS -1,11; J20.MA_DATA[2] 0,11; J21.MA_DATA[13] 1,11; J22.VSS 2,11; J23.MA_DM[1] 3,11; J24.MA_DATA[11] 4,11; J25.VSS 5,11; J26.MA_DATA[16] 6,11; J27.MA_DATA[17] 7,11; J28.VSS 8,11; J29.MA_DATA[28] 9,11; J30.MA_DATA[25] 10,11; J31.VSS 11,11; J32.MA_CHECK[6] 12,11; J33.MA_CHECK[7] 13,11; J34.VSS 14,11; J35.VSS 15,11; J36.RSVD 16,11; J37.VSS 17,11; J38.RSVD 18,11; J39.MB_CHECK[3] 19,11; K1.P_GFX_TXP[6] -19,10; K2.P_GFX_TXN[5] -18,10; K3.VDDCR_SOC -17,10; K4.P_GFX_RXN[5] -16,10; K5.P_GFX_RXP[5] -15,10; K6.VDDCR_SOC -14,10; K7.P_GFX_RXN[4] -13,10; K8.P_GFX_RXP[4] -12,10; K9.VDDCR_SOC -11,10; K10.VSS -10,10; K11.VDDCR_SOC -9,10; K12.VSS -8,10; K13.VDDCR_SOC -7,10; K14.DP_STEREOSYNC -6,10; K15.VDDCR_SOC -5,10; K18.VSS -2,10; K19.MA_DM[0] -1,10; K20.VSS 0,10; K21.VSS 1,10; K22.VSS 2,10; K23.VSS 3,10; K26.VSS 6,10; K27.VSS 7,10; K28.VSS 8,10; K29.VSS 9,10; K30.VSS 10,10; K31.MA_CHECK[2] 11,10; K32.MA_CHECK[3] 12,10; K33.VSS 13,10; K34.RSVD 14,10; K35.MB_RESET_L 15,10; K36.VDDIO_MEM_S3 16,10; K37.MB0_CKE[1] 17,10; K38.RSVD 18,10; K39.VDDIO_MEM_S3 19,10; L2.VDDCR_SOC -18,9; L3.P_GFX_TXP[7] -17,9; L4.VSS -16,9; L5.VSS -15,9; L6.P_GFX_RXN[6] -14,9; L7.P_GFX_RXP[6] -13,9; L8.VSS -12,9; L9.VSS -11,9; L10.VDDCR_SOC -10,9; L11.VSS -9,9; L12.VDDCR_SOC -8,9; L13.VSS -7,9; L14.VDDCR_SOC -6,9; L15.VSS -5,9; L16.VDDCR_SOC -4,9; L17.VSS -3,9; L18.VDDCR_SOC -2,9; L19.VSS -1,9; L20.VDDCR_SOC 0,9; L21.VSS 1,9; L22.VDDCR_SOC 2,9; L23.TEST4 3,9; L24.VDDCR_SOC 4,9; L25.VSS 5,9; L26.VDDCR_SOC 6,9; L27.VSS 7,9; L28.VSS 8,9; L29.VSS 9,9; L30.VSS 10,9; L31.VSS 11,9; L32.VDDIO_MEM_S3 12,9; L33.MA_RESET_L 13,9; L34.MA1_CKE[1] 14,9; L35.VDDIO_MEM_S3 15,9; L36.MB1_CKE[1] 16,9; L37.MB0_CKE[0] 17,9; L38.VDDIO_MEM_S3 18,9; L39.MB1_CKE[0] 19,9; M2.P_GFX_TXP[8] -18,8; M3.P_GFX_TXN[7] -17,8; M4.VSS -16,8; M5.P_GFX_RXN[7] -15,8; M6.P_GFX_RXP[7] -14,8; M7.VDDCR_CPU -13,8; M8.VSS -12,8; M9.VDDCR_SOC -11,8; M10.VSS -10,8; M11.VDDCR_SOC -9,8; M12.VSS -8,8; M13.VDDCR_SOC -7,8; M14.VSS -6,8; M15.VDDCR_SOC -5,8; M16.VSS -4,8; M17.VDDCR_SOC -3,8; M18.VSS -2,8; M19.VDDCR_SOC -1,8; M20.VSS 0,8; M21.VDDCR_SOC 1,8; M22.TEST5 2,8; M23.VDDCR_SOC 3,8; M24.VSS 4,8; M25.VDDCR_SOC 5,8; M26.VSS 6,8; M27.VSS 7,8; M28.VSS 8,8; M29.VDDIO_MEM_S3 9,8; M30.MA0_CKE[1] 10,8; M31.VDDIO_MEM_S3 11,8; M32.MA0_CKE[0] 12,8; M33.MA1_CKE[0] 13,8; M34.VDDIO_MEM_S3 14,8; M35.MA_ACT_L 15,8; M36.MB_BG[0] 16,8; M37.VDDIO_MEM_S3 17,8; M38.MB_ACT_L 18,8; M39.MB_BG[1] 19,8; N2.P_GFX_TXN[8] -18,7; N3.VDDCR_CPU -17,7; N4.P_GFX_RXN[9] -16,7; N5.P_GFX_RXP[9] -15,7; N6.VDDCR_CPU -14,7; N7.P_GFX_RXN[8] -13,7; N8.P_GFX_RXP[8] -12,7; N9.VSS -11,7; N10.VDDCR_SOC -10,7; N11.VSS -9,7; N12.VDDCR_SOC -8,7; N13.VSS -7,7; N14.VDDCR_SOC -6,7; N15.VSS -5,7; N16.VDDCR_SOC -4,7; N17.VSS -3,7; N18.VDDCR_SOC -2,7; N19.VSS -1,7; N20.VDDCR_SOC 0,7; N21.VSS 1,7; N22.VDDCR_SOC 2,7; N23.VSS 3,7; N24.VDDCR_SOC 4,7; N25.VSS 5,7; N26.VDDCR_SOC 6,7; N27.VSS 7,7; N28.VDDIO_MEM_S3 8,7; N29.VSS 9,7; N30.VDDIO_MEM_S3 10,7; N31.MA_BG[0] 11,7; N32.MA_BG[1] 12,7; N33.VDDIO_MEM_S3 13,7; N34.MA_ALERT_L 14,7; N35.MA_ADD[12] 15,7; N36.VDDIO_MEM_S3 16,7; N37.MB_ALERT_L 17,7; N38.MB_ADD[12] 18,7; N39.VDDIO_MEM_S3 19,7; P1.P_GFX_TXN[9] -19,6; P2.VDDCR_CPU -18,6; P3.P_GFX_TXP[10] -17,6; P4.VSS -16,6; P5.VSS -15,6; P6.P_GFX_RXN[10] -14,6; P7.P_GFX_RXP[10] -13,6; P8.VSS -12,6; P9.VDDCR_SOC -11,6; P10.VSS -10,6; P11.VDDCR_SOC -9,6; P12.VSS -8,6; P13.VDDCR_SOC -7,6; P27.VDDIO_MEM_S3 7,6; P28.TEST47 8,6; P29.VDDIO_MEM_S3 9,6; P30.MA_ADD[8] 10,6; P31.MA_ADD[9] 11,6; P32.VDDIO_MEM_S3 12,6; P33.MA_ADD[11] 13,6; P34.MA_ADD[7] 14,6; P35.VDDIO_MEM_S3 15,6; P36.MB_ADD[9] 16,6; P37.MB_ADD[11] 17,6; P38.VDDIO_MEM_S3 18,6; P39.MB_ADD[7] 19,6; R1.VSS -19,5; R2.P_GFX_TXP[11] -18,5; R3.P_GFX_TXN[10] -17,5; R4.VSS -16,5; R5.P_GFX_RXN[11] -15,5; R6.P_GFX_RXP[11] -14,5; R7.VDDCR_CPU -13,5; R8.VSS -12,5; R9.VSS -11,5; R10.VDDCR-SOC -10,5; R11.VSS -9,5; R12.VDDCR_SOC -8,5; R13.VSS -7,5; R27.VSS 7,5; R28.VDDIO_MEM_S3 8,5; R29.VSS 9,5; R30.MA_ADD[4] 10,5; R31.VDDIO_MEM_S3 11,5; R32.MA_ADD[6] 12,5; R33.MA_ADD[5] 13,5; R34.VDDIO_MEM_S3 14,5; R35.RSVD 15,5; R36.MB_ADD[6] 16,5; R37.VDDIO_MEM_S3 17,5; R38.MB_ADD[8] 18,5; R39.MB_ADD[5] 19,5; T1.P_GFX_TXP[12] -19,4; T2.P_GFX_TXN[11] -18,4; T3.VDDCR_CPU -17,4; T4.P_GFX_RXP[13] -16,4; T5.P_GFX_RXN[13] -15,4; T6.VDDCR_CPU -14,4; T7.P_GFX_RXN[12] -13,4; T8.P_GFX_RXP[12] -12,4; T9.VDDCR_CPU -11,4; T10.VSS -10,4; T11.VDDCR_SOC -9,4; T12.VSS -8,4; T13.VDDCR_SOC -7,4; T27.VDDIO_MEM_S3 7,4; T28.VSS 8,4; T29.VDDIO_MEM_S3 9,4; T30.VSS 10,4; T31.MA_ADD[3] 11,4; T32.MA_ADD[1] 12,4; T33.VDDIO_MEM_S3 13,4; T34.MA_CLK_H[0] 14,4; T35.MA_ADD[2] 15,4; T36.VDDIO_MEM_S3 16,4; T37.MB_ADD[4] 17,4; T38.MB_ADD[3] 18,4; T39.VDDIO_MEM_S3 19,4; U1.P_GFX_TXN[12] -19,3; U2.VDDCR_CPU -18,3; U3.P_GFX_TXP[13] -17,3; U4.VSS -16,3; U5.VSS -15,3; U6.P_GFX_RXN[14] -14,3; U7.P_GFX_RXP[14] -13,3; U8.VSS -12,3; U9.VSS -11,3; U10.VDDCR_CPU -10,3; U11.VSS -9,3; U12.VDDCR_SOC -8,3; U13.VSS -7,3; U27.VSS 7,3; U28.VDDIO_MEM_S3 8,3; U29.VSS 9,3; U30.VDDIO_MEM_S3 10,3; U31.VSS 11,3; U32.VDDIO_MEM_S3 12,3; U33.MA_CLK_H[1] 13,3; U34.MA_CLK_L[0] 14,3; U35.VDDIO_MEM_S3 15,3; U36.MB_ADD[1] 16,3; U37.MB_ADD[2] 17,3; U38.VDDIO_MEM_S3 18,3; U39.MB_CLK_H[0] 19,3; V1.VSS -19,2; V2.P_GFX_TXP[14] -18,2; V3.P_GFX_TXN[13] -17,2; V4.VSS -16,2; V5.P_GFX_RXN[15] -15,2; V6.P_GFX_RXP[15] -14,2; V7.VSS -13,2; V8.P0A_ZVSS -12,2; V9.VDDCR_CPU -11,2; V10.VSS -10,2; V11.VDDCR_CPU -9,2; V12.VSS -8,2; V13.VDDCR_SOC -7,2; V27.VDDIO_MEM_S3 7,2; V28.VSS 8,2; V29.VDDIO_MEM_S3 9,2; V30.VSS 10,2; V31.VDDIO_MEM_S3 11,2; V32.MA_CLK_H[3] 12,2; V33.MA_CLK_L[1] 13,2; V34.VDDIO_MEM_S3 14,2; V35.MA_CLK_H[2] 15,2; V36.MA_CLK_L[2] 16,2; V37.VDDIO_MEM_S3 17,2; V38.MB_CLK_H[1] 18,2; V39.MB_CLK_L[0] 19,2; W1.P_GFX_TXP[15] -19,1; W2.P_GFX_TXN[14] -18,1; W3.VDDCR_CPU -17,1; W4.P_HUB_RXP[3] -16,1; W5.P_HUB_RXN[3] -15,1; W6.VDDCR_CPU -14,1; W7.P_ZVSS -13,1; W8.P_ZVDDP -12,1; W9.VSS -11,1; W10.VDDCR_CPU -10,1; W11.VSS -9,1; W12.VDDCR_CPU -8,1; W13.VSS -7,1; W27.VSS 7,1; W28.VDDIO_MEM_S3 8,1; W29.VSS 9,1; W30.TEST40 10,1; W31.VSS 11,1; W32.MA_CLK_L[3] 12,1; W33.VDDIO_MEM_S3 13,1; W34.VDDIO_MEM_S3 14,1; W35.MA_EVENT_L 15,1; W36.VDDIO_MEM_S3 16,1; W37.MB_CLK_H[2] 17,1; W38.MB_CLK_L[1] 18,1; W39.VDDIO_MEM_S3 19,1; Y1.P_GFX_TXN[15] -19,0; Y2.VDDCR_CPU -18,0; Y3.USB_SS_0RXP -17,0; Y4.USB_SS_0RXN -16,0; Y5.VSS -15,0; Y6.P_HUB_RXP[2] -14,0; Y7.P_HUB_RXN[2] -13,0; Y8.VSS -12,0; Y9.VDDCR_CPU -11,0; Y10.VSS -10,0; Y11.VDDCR_CPU -9,0; Y12.VSS -8,0; Y13.VDDCR_CPU -7,0; Y27.VDDIO_MEM_S3 7,0; Y28.VSS 8,0; Y29.VDDIO_MEM_S3 9,0; Y30.VSS 10,0; Y31.VDDIO_MEM_S3 11,0; Y32.VDDIO_MEM_S3 12,0; Y33.MA_PARTOUT 13,0; Y34.MA__ZVDDIO_MEM_S3 14,0; Y35.VDDIO_MEM_S3 15,0; Y36.MB__ZVDDIO_MEM_S3 16,0; Y37.MB_CLK_L[2] 17,0; Y38.VDDIO_MEM_S3 18,0; Y39.MB_CLK_H[3] 19,0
